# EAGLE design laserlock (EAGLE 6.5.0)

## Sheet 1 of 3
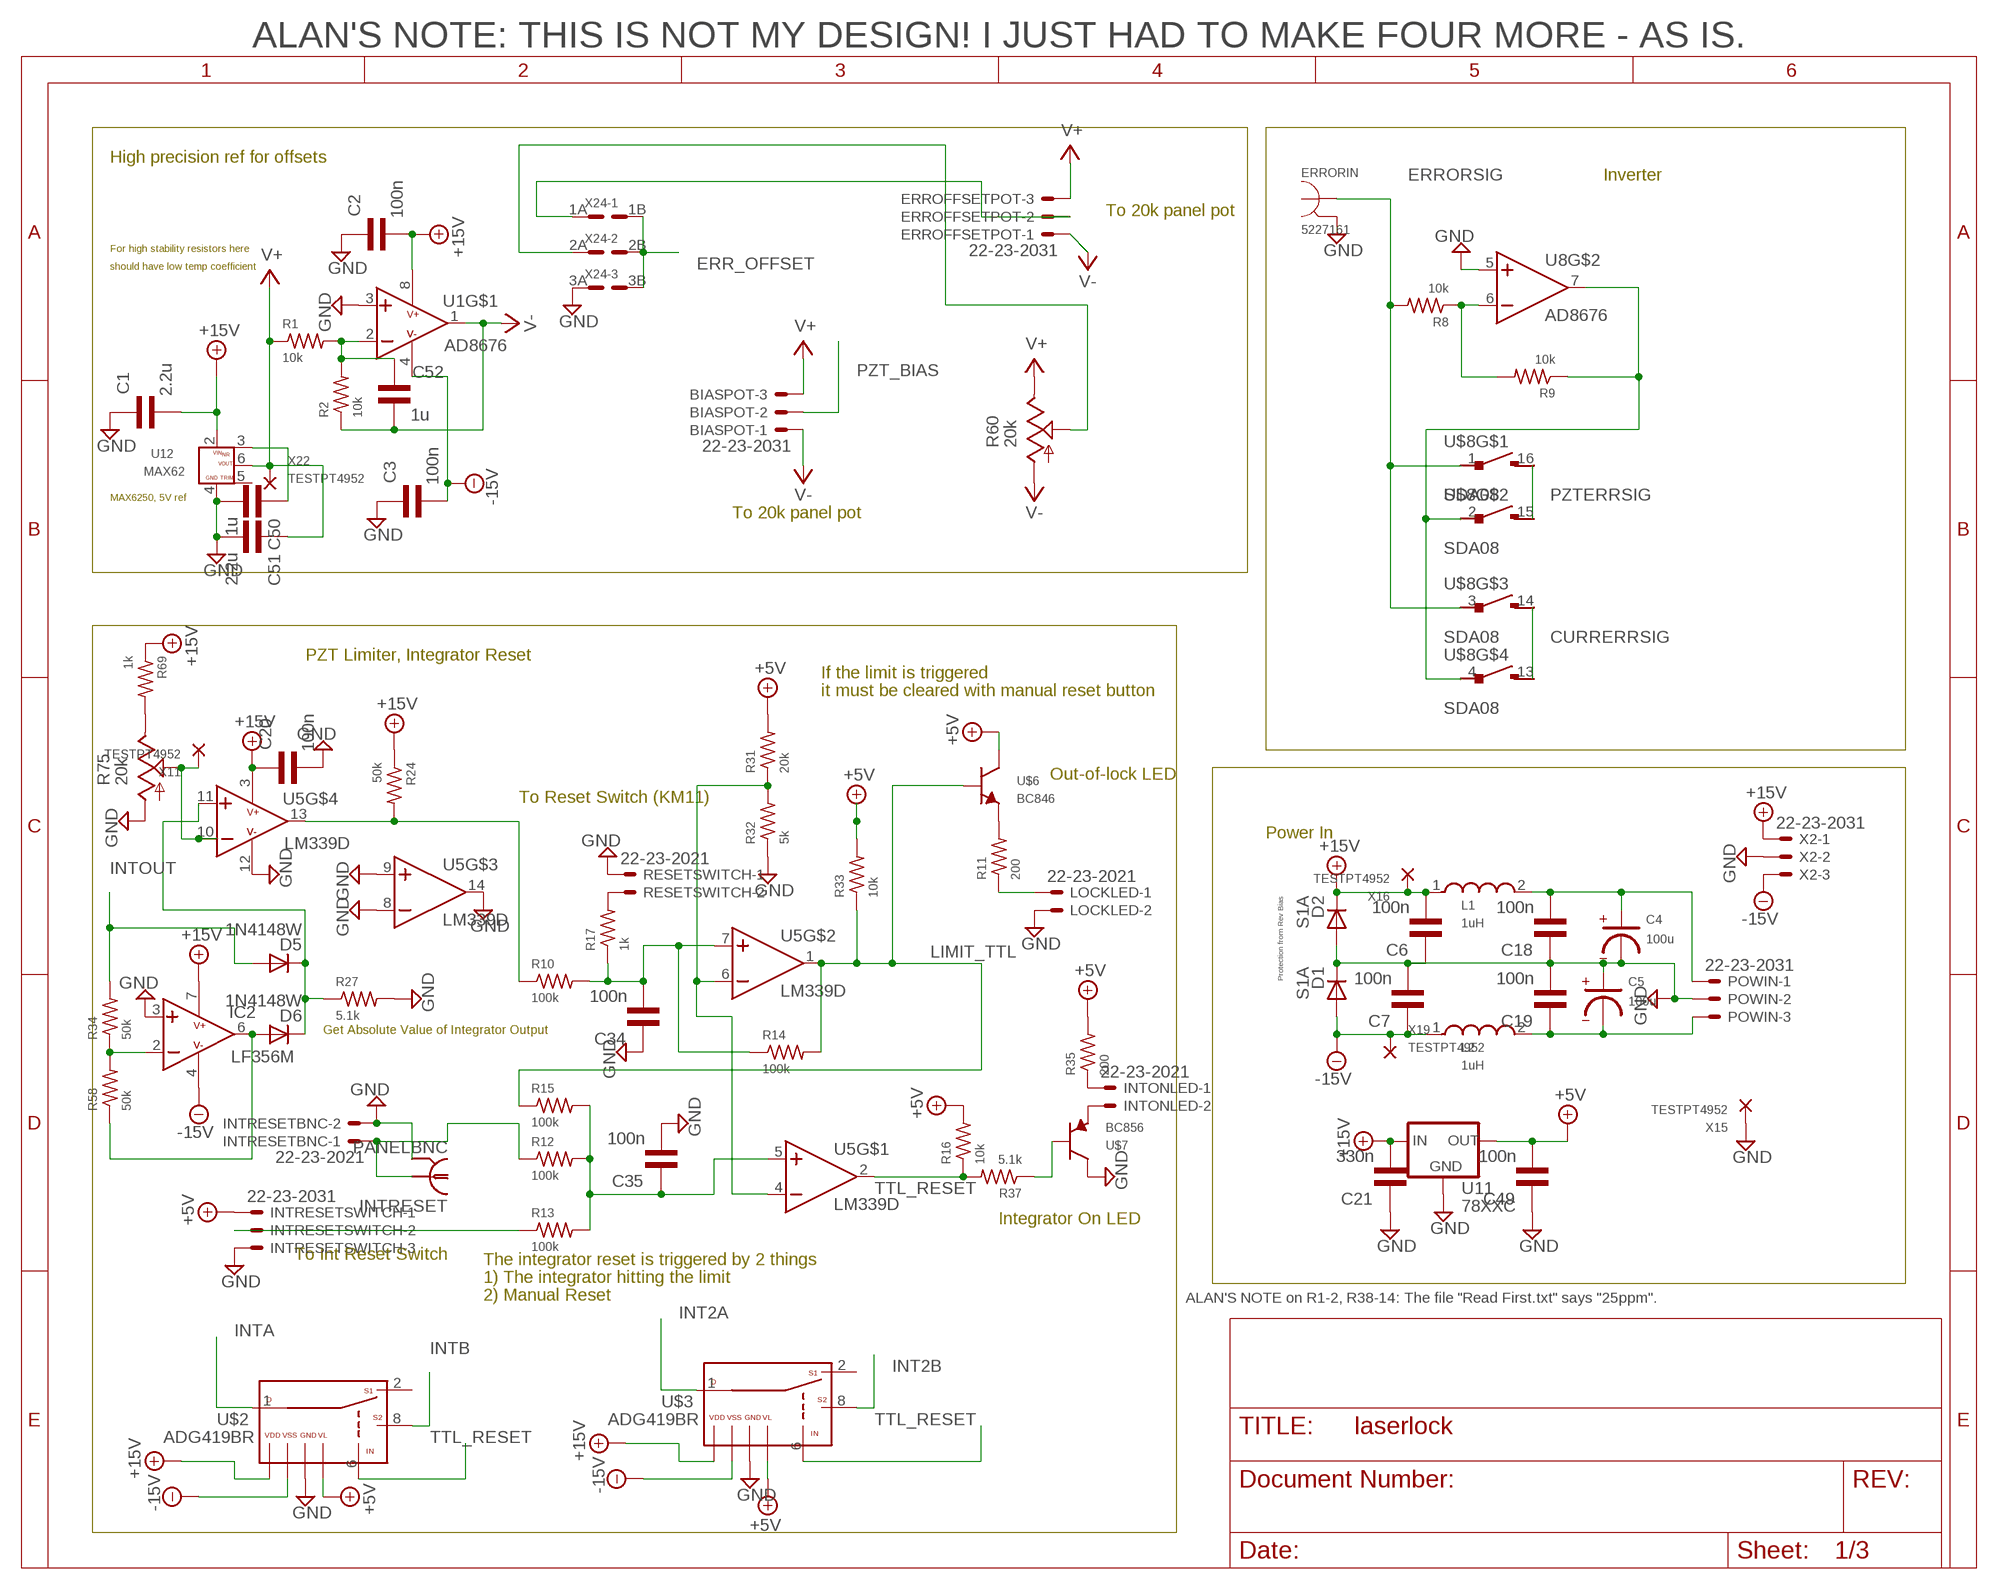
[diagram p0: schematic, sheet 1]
INTRESET (PANELBNC): DISTRIBUTOR: L-COM; PARTNUM: BAC1503

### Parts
BIASPOT  22-23-2031  [22-23-2031]
C1  2.2u  CAP0805  [0805]
C2  100n  CAP0805  [0805]
C3  100n  CAP0805  [0805]
C4  100u  CAPPOLRADIAL-0.1SPACING  [ELECCAPTH1]
C5  100u  CAPPOLRADIAL-0.1SPACING  [ELECCAPTH1]
C6  100n  CAP0805  [0805]
C7  100n  CAP0805  [0805]
C18  100n  CAP0805  [0805]
C19  100n  CAP0805  [0805]
C20  100n  CAP0805  [0805]
C21  330n  CAP0805  [0805]
C34  100n  CAP0805  [0805]
C35  100n  CAP0805  [0805]
C49  100n  CAP0805  [0805]
C50  1u  CAP0805  [0805]
C51  2.2u  CAP0805  [0805]
C52  1u  CAP0805  [0805]
D1  S1A  [DO-214AC]
D2  S1A  [DO-214AC]
D5  1N4148W  [SOD-323F]
D6  1N4148W  [SOD-323F]
ERROFFSETPOT  22-23-2031  [22-23-2031]
ERRORIN  5227161  [5227161]
IC2  LF356M  [SO08]
INTONLED  22-23-2021  [22-23-2021]
INTRESETBNC  22-23-2021  [22-23-2021]
INTRESETSWITCH  22-23-2031  [22-23-2031]
L1  1uH  INDUCTOR0805  [0805]
L2  1uH  INDUCTOR0805  [0805]
LOCKLED  22-23-2021  [22-23-2021]
POWIN  22-23-2031  [22-23-2031]
R1  10k  RESISTOR0805  [0805]
R2  10k  RESISTOR0805  [0805]
R8  10k  RESISTOR0805  [0805]
R9  10k  RESISTOR0805  [0805]
R10  100k  RESISTOR0805  [0805]
R11  200  RESISTOR1210  [1210]
R12  100k  RESISTOR0805  [0805]
R13  100k  RESISTOR0805  [0805]
R14  100k  RESISTOR0805  [0805]
R15  100k  RESISTOR0805  [0805]
R16  10k  RESISTOR0805  [0805]
R17  1k  RESISTOR0805  [0805]
R24  50k  RESISTOR0805  [0805]
R27  5.1k  RESISTOR0805  [0805]
R31  20k  RESISTOR0805  [0805]
R32  5k  RESISTOR0805  [0805]
R33  10k  RESISTOR0805  [0805]
R34  50k  RESISTOR0805  [0805]
R35  200  RESISTOR1210  [1210]
R37  5.1k  RESISTOR0805  [0805]
R58  50k  RESISTOR0805  [0805]
R60  20k  BITECH23B  [BITECH23B]
R69  1k  RESISTOR0805  [0805]
R75  20k  BITECH23B  [BITECH23B]
RESETSWITCH  22-23-2021  [22-23-2021]
U1  AD8676  [SO08]
U5  LM339D  [SO14]
U8  AD8676  [SO08]
U11  78XXC  [TO-220]
U12  MAX62  [SO08]
U$2  ADG419BR  [SO08]
U$3  ADG419BR  [SO08]
U$6  BC846  [SOT-23]
U$7  BC856  [SOT-23]
U$8  SDA08  [DIL16]
X2  22-23-2031  [22-23-2031]
X11  TESTPT4952  [TESTPT4952]
X15  TESTPT4952  [TESTPT4952]
X16  TESTPT4952  [TESTPT4952]
X19  TESTPT4952  [TESTPT4952]
X22  TESTPT4952  [TESTPT4952]
X24  HEADER2ROW3POS  [HEADER2ROW3POS]

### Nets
+5V: C49.2 INTRESETSWITCH.1 R16.2 R31.2 R33.2 R35.P$2 U11.3(OUT) U$2.5(VL) U$3.5(VL) U$6.3(C)
+15V: C1.2 C2.2 C6.2 C20.1 C21.2 D2.1(CATHODE) IC2.7(V+) L1.1 R24.1 R69.1 U1.8(V+) U5.3(V+) U11.1(IN) U12.2(VIN) U$2.4(V+) U$3.4(V+) X2.1 X16.P$1 ; also sheet 2,3
-15V: C3.2 C7.1 D1.2(ANODE) IC2.4(V-) L2.1 U1.4(V-) U$2.7(V-) U$3.7(V-) X2.3 X19.P$1 ; also sheet 2,3
CURRERRSIG: U$8.13 U$8.14 ; also sheet 3
ERR_OFFSET: X24.1B X24.2B X24.3B ; also sheet 2
ERRORSIG: ERRORIN.INCOND R8.2 U$8.1 U$8.3
GND: C1.1 C2.1 C3.1 C4.MINUS C5.PLUS C6.1 C7.2 C18.1 C19.2 C20.2 C21.1 C34.1 C35.2 C49.1 C50.2 C51.2 D1.1(CATHODE) D2.2(ANODE) ERRORIN.OUTCOND IC2.3(IN+) INTRESETBNC.2 INTRESETSWITCH.3 LOCKLED.2 POWIN.2 R27.2 R32.1 R75.1(A) RESETSWITCH.1 U1.3(IN+) U5.8(IN-) U5.9(IN+) U5.12(V-) U5.14(OUT) U8.5(IN+) U11.2(GND) U12.4(GND) U$2.3(GND) U$3.3(GND) U$7.3(C) X2.2 X15.P$1 X24.3A ; also sheet 2,3
INT2A: U$3.1(D) ; also sheet 2
INT2B: U$3.8(S2) ; also sheet 2
INTA: U$2.1(D) ; also sheet 2
INTB: U$2.8(S2) ; also sheet 2
INTOUT: D5.1(ANODE) R34.2 ; also sheet 2
LIMIT_TTL: R14.2 R15.1 R33.1 U5.1(OUT) U$6.1(B)
N$2: C52.1 R1.2 R2.2 U1.2(IN-)
N$5: R69.2 R75.3(E)
N$10: INTRESETBNC.1 R12.1
N$11: INTONLED.2 U$7.2(E)
N$12: INTRESETSWITCH.2 R13.1
N$13: R37.1 U$7.1(B)
N$14: C50.1 U12.3(NR)
N$15: R8.1 R9.2 U8.6(IN-)
N$16: C34.2 R10.2 R14.1 R17.1 U5.7(IN+)
N$17: C35.1 R12.2 R13.2 R15.2 U5.5(IN+)
N$18: R17.2 RESETSWITCH.2
N$37: ERROFFSETPOT.2 X24.1A
N$39: R9.1 U8.7(OUT) U$8.2 U$8.4
N$40: R10.1 R24.2 U5.13(OUT)
N$41: R31.1 R32.2 U5.4(IN-) U5.6(IN-)
N$42: R11.P$2 U$6.2(E)
N$43: R75.2(S) U5.10(IN-) X11.P$1
N$45: LOCKLED.1 R11.P$1
N$49: C5.MINUS C19.1 L2.2 POWIN.3
N$50: C4.PLUS C18.2 L1.2 POWIN.1
N$51: D5.2(CATHODE) D6.2(CATHODE) R27.1 U5.11(IN+)
N$54: R60.2(S) X24.2A
N$70: INTONLED.1 R35.P$1
N$80: IC2.2(IN-) R34.1 R58.2
N$81: D6.1(ANODE) IC2.6(OUT) R58.1
PZT_BIAS: BIASPOT.2 ; also sheet 2
PZTERRSIG: U$8.15 U$8.16 ; also sheet 2
TTL_RESET: R16.1 R37.2 U5.2(OUT) U$2.6(IN) U$3.6(IN)
V+: BIASPOT.3 C51.1 ERROFFSETPOT.3 R1.1 R60.3(E) U12.6(VO) X22.P$1
V-: BIASPOT.1 C52.2 ERROFFSETPOT.1 R2.1 R60.1(A) U1.1(OUT)
Unconnected: U12.5(TRIM) U$2.2(S1) U$3.2(S1)

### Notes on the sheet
- ALAN'S NOTE: THIS IS NOT MY DESIGN! I JUST HAD TO MAKE FOUR MORE - AS IS.
- High precision ref for offsets
- Inverter
- To 20k panel pot
- For high stability resistors here
- should have low temp coefficient
- MAX6250, 5V ref
- To 20k panel pot
- PZT Limiter, Integrator Reset
- If the limit is triggered
- it must be cleared with manual reset button
- Out-of-lock LED
- To Reset Switch (KM11)
- Power In
- Protection from Rev Bias
- Get Absolute Value of Integrator Output
- Integrator On LED
- To Int Reset Switch
- The integrator reset is triggered by 2 things
- 1) The integrator hitting the limit
- ALAN'S NOTE on R1-2, R38-14: The file "Read First.txt" says "25ppm".
- 2) Manual Reset

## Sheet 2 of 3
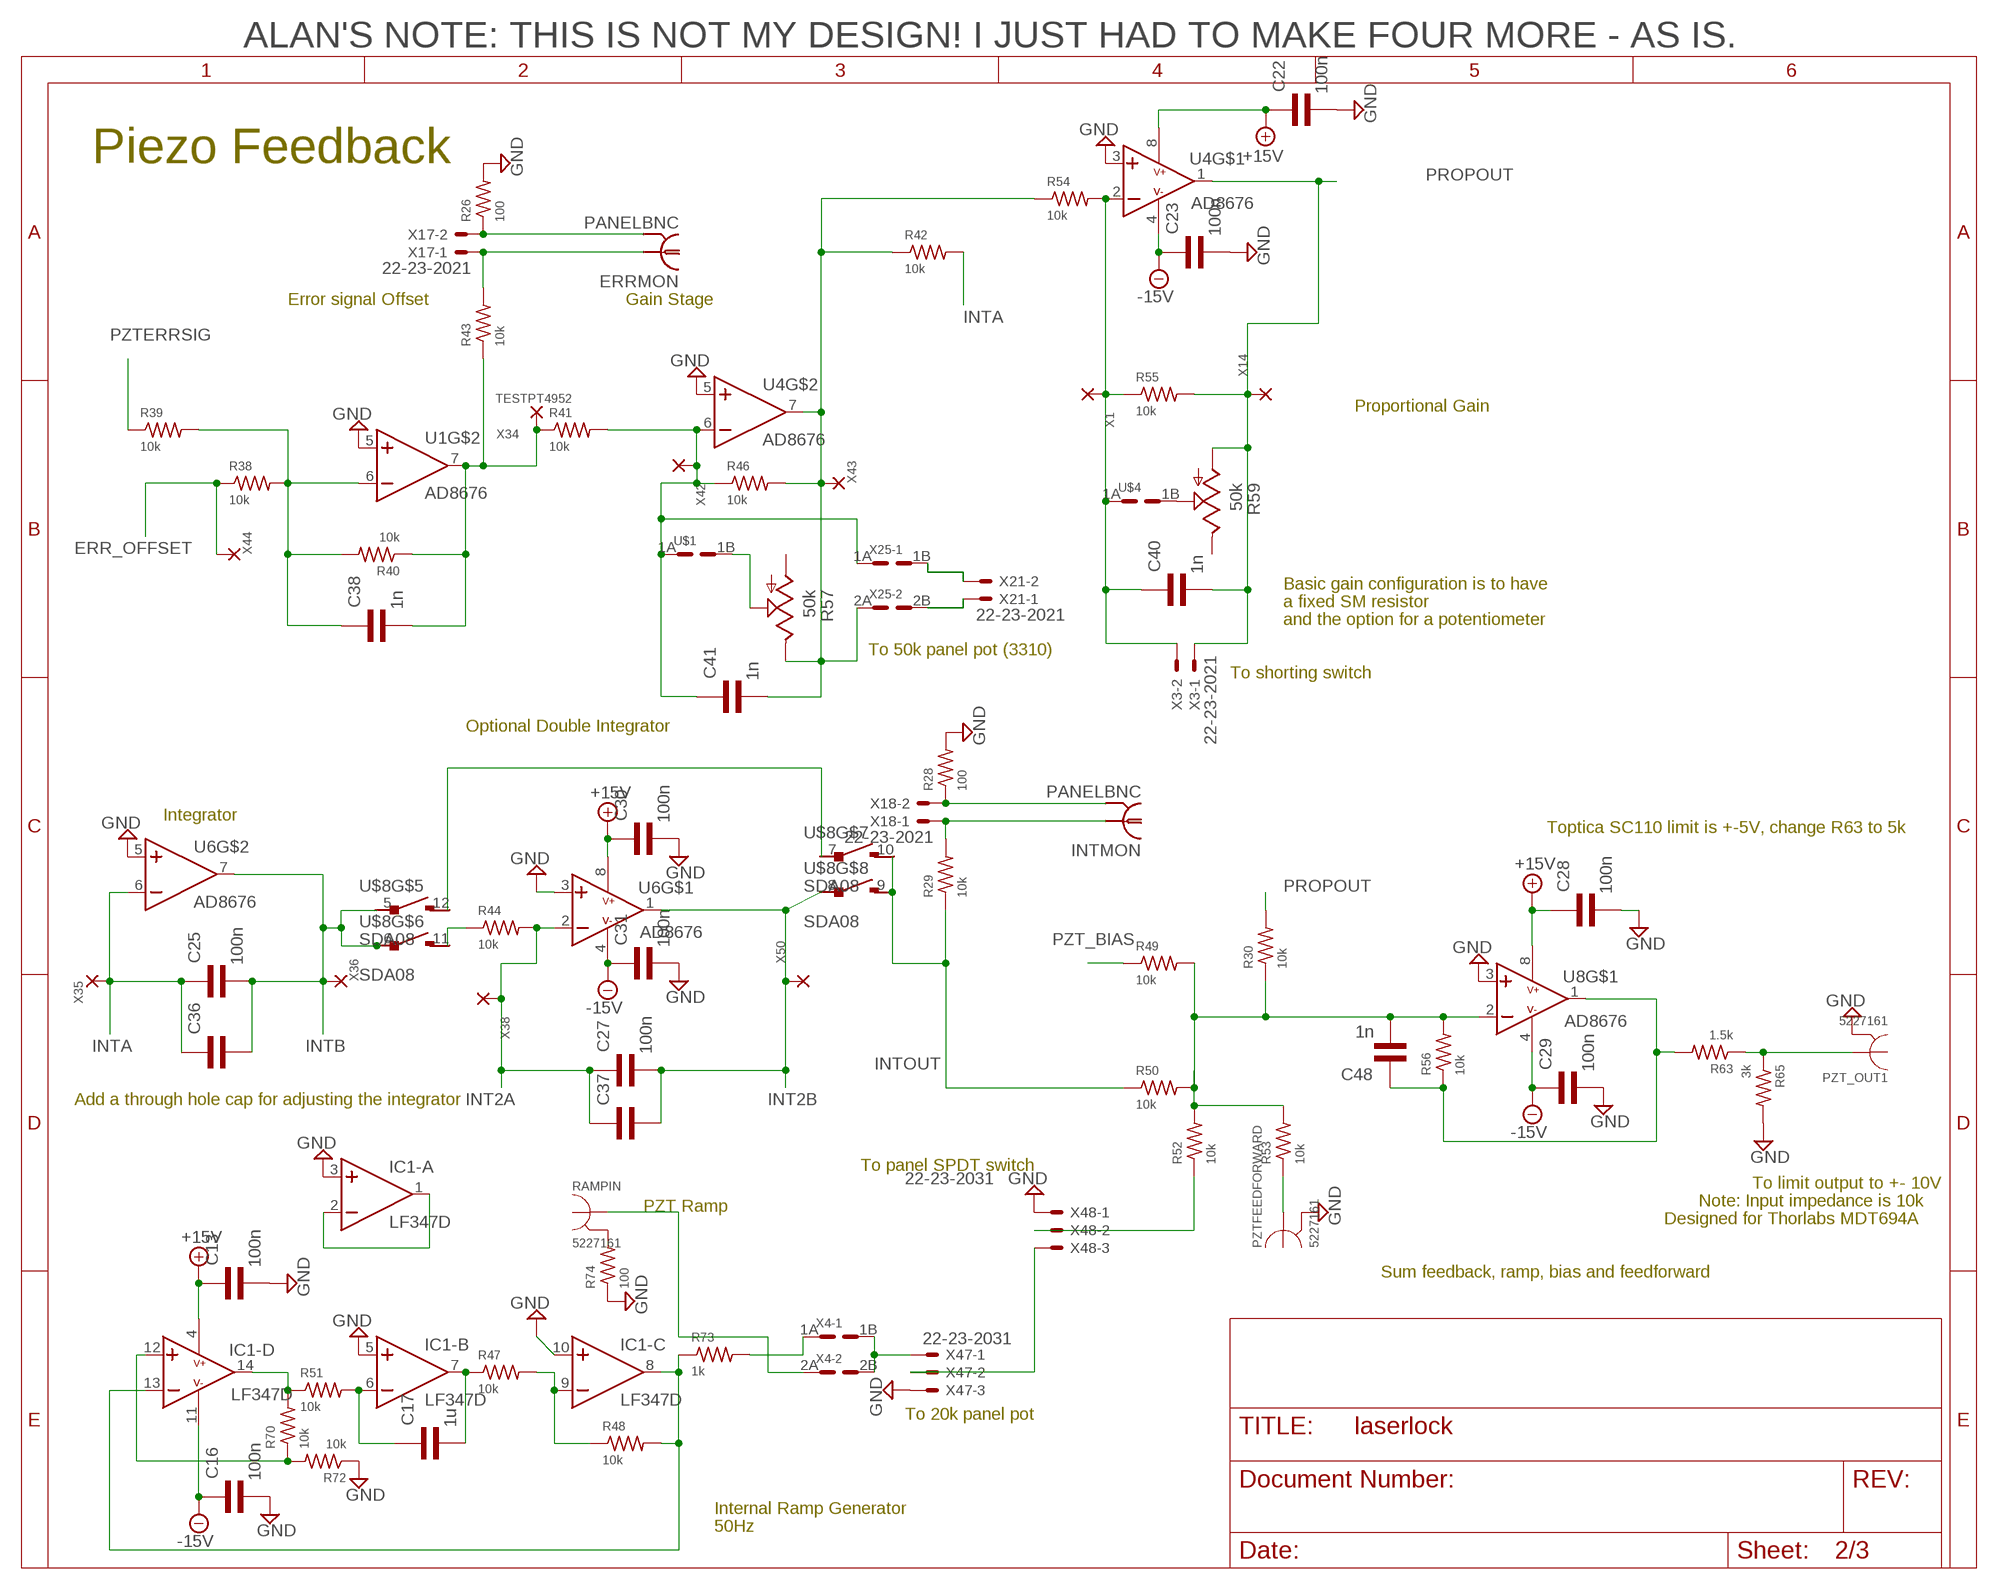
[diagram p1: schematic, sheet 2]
ERRMON (PANELBNC): DISTRIBUTOR: L-COM; PARTNUM: BAC1503
INTMON (PANELBNC): DISTRIBUTOR: L-COM; PARTNUM: BAC1503

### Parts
C13  100n  CAP0805  [0805]
C16  100n  CAP0805  [0805]
C17  1u  CAP0805  [0805]
C22  100n  CAP0805  [0805]
C23  100n  CAP0805  [0805]
C25  100n  CAP0805  [0805]
C27  100n  CAP0805  [0805]
C28  100n  CAP0805  [0805]
C29  100n  CAP0805  [0805]
C30  100n  CAP0805  [0805]
C31  100n  CAP0805  [0805]
C36  CAPTH1  [TH1]
C37  CAPTH1  [TH1]
C38  1n  CAP0805  [0805]
C40  1n  CAP0805  [0805]
C41  1n  CAP0805  [0805]
C48  1n  CAP0805  [0805]
IC1  LF347D  [SO14]
PZT_OUT1  5227161  [5227161]
PZTFEEDFORWARD  5227161  [5227161]
R26  100  RESISTOR0805  [0805]
R28  100  RESISTOR0805  [0805]
R29  10k  RESISTOR0805  [0805]
R30  10k  RESISTOR0805  [0805]
R38  10k  RESISTOR0805  [0805]
R39  10k  RESISTOR0805  [0805]
R40  10k  RESISTOR0805  [0805]
R41  10k  RESISTOR0805  [0805]
R42  10k  RESISTOR0805  [0805]
R43  10k  RESISTOR0805  [0805]
R44  10k  RESISTOR0805  [0805]
R46  10k  RESISTOR0805  [0805]
R47  10k  RESISTOR0805  [0805]
R48  10k  RESISTOR0805  [0805]
R49  10k  RESISTOR0805  [0805]
R50  10k  RESISTOR0805  [0805]
R51  10k  RESISTOR0805  [0805]
R52  10k  RESISTOR0805  [0805]
R53  10k  RESISTOR0805  [0805]
R54  10k  RESISTOR0805  [0805]
R55  10k  RESISTOR0805  [0805]
R56  10k  RESISTOR0805  [0805]
R57  50k  BITECH23B  [BITECH23B]
R59  50k  BITECH23B  [BITECH23B]
R63  1.5k  RESISTOR0805  [0805]
R65  3k  RESISTOR0805  [0805]
R70  10k  RESISTOR0805  [0805]
R72  10k  RESISTOR0805  [0805]
R73  1k  RESISTOR0805  [0805]
R74  100  RESISTOR0805  [0805]
RAMPIN  5227161  [5227161]
U4  AD8676  [SO08]
U6  AD8676  [SO08]
U$1  HEADER2ROW1POS  [HEADER2ROW1POS]
U$4  HEADER2ROW1POS  [HEADER2ROW1POS]
X1  TESTPT4952  [TESTPT4952]
X3  22-23-2021  [22-23-2021]
X4  HEADER2ROW2POS  [HEADER2ROW2POS]
X14  TESTPT4952  [TESTPT4952]
X17  22-23-2021  [22-23-2021]
X18  22-23-2021  [22-23-2021]
X21  22-23-2021  [22-23-2021]
X25  HEADER2ROW2POS  [HEADER2ROW2POS]
X34  TESTPT4952  [TESTPT4952]
X35  TESTPT4952  [TESTPT4952]
X36  TESTPT4952  [TESTPT4952]
X38  TESTPT4952  [TESTPT4952]
X42  TESTPT4952  [TESTPT4952]
X43  TESTPT4952  [TESTPT4952]
X44  TESTPT4952  [TESTPT4952]
X47  22-23-2031  [22-23-2031]
X48  22-23-2031  [22-23-2031]
X50  TESTPT4952  [TESTPT4952]

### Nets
+15V: C13.1 C22.1 C28.1 C30.1 IC1.4(-D:V+) U4.8(V+) U6.8(V+) U8.8(V+) ; also sheet 1,3
-15V: C16.1 C23.1 C29.1 C31.1 IC1.11(-D:V-) U4.4(V-) U6.4(V-) U8.4(V-) ; also sheet 1,3
ERR_OFFSET: R38.1 X44.P$1 ; also sheet 1
GND: C13.2 C16.2 C22.2 C23.2 C28.2 C29.2 C30.2 C31.2 IC1.3(-A:IN+) IC1.5(-B:IN+) IC1.10(-C:IN+) PZT_OUT1.OUTCOND PZTFEEDFORWARD.OUTCOND R26.2 R28.2 R65.2 R72.1 R74.1 U1.5(IN+) U4.3(IN+) U4.5(IN+) U6.3(IN+) U6.5(IN+) U8.3(IN+) X47.3 X48.1 ; also sheet 1,3
INT2A: C27.1 C37.P$1 R44.2 U6.2(IN-) X38.P$1 ; also sheet 1
INT2B: C27.2 C37.P$2 U6.1(OUT) U$8.8 X50.P$1 ; also sheet 1
INTA: C25.1 C36.P$1 R42.2 U6.6(IN-) X35.P$1 ; also sheet 1
INTB: C25.2 C36.P$2 U6.7(OUT) U$8.5 U$8.6 X36.P$1 ; also sheet 1
INTOUT: R29.1 R50.1 U$8.9 U$8.10 ; also sheet 1
N$21: C41.2 R42.1 R46.2 R54.1 R57.3(E) U4.7(OUT) X25.2A X43.P$1
N$28: R26.1 X17.2
N$29: R29.2 X18.1
N$30: X21.2 X25.1B
N$33: IC1.1(-A:OUT) IC1.2(-A:IN-)
N$34: C17.2 IC1.7(-B:OUT) R47.1
N$35: R43.2 X17.1
N$36: R28.1 X18.2
N$38: X21.1 X25.2B
N$46: C40.1 R54.2 R55.1 U4.2(IN-) U$4.1A X1.P$1 X3.2
N$47: C38.1 R38.2 R39.2 R40.2 U1.6(IN-)
N$48: C38.2 R40.1 R41.1 R43.1 U1.7(OUT) X34.P$1
N$53: U$8.7 U$8.12
N$55: R44.1 U$8.11
N$56: X47.2 X48.3
N$59: C41.1 R41.2 R46.1 U4.6(IN-) U$1.1A X25.1A X42.P$1
N$60: R57.2(S) U$1.1B
N$62: IC1.9(-C:IN-) R47.2 R48.1
N$63: IC1.8(-C:OUT) IC1.13(-D:IN-) R48.2 R73.1
N$64: C17.1 IC1.6(-B:IN-) R51.2
N$65: X4.1B X4.2B X47.1
N$66: R59.2(S) U$4.1B
N$67: PZTFEEDFORWARD.INCOND R53.1
N$68: C48.2 R30.1 R49.2 R50.2 R52.2 R53.2 R56.2 U8.2(IN-)
N$69: R52.1 X48.2
N$72: C48.1 R56.1 R63.2 U8.1(OUT)
N$73: PZT_OUT1.INCOND R63.1 R65.1
N$75: IC1.14(-D:OUT) R51.1 R70.2
N$78: IC1.12(-D:IN+) R70.1 R72.2
N$82: RAMPIN.INCOND X4.2A
N$83: R73.2 X4.1A
N$84: R74.2 RAMPIN.OUTCOND
PROPOUT: C40.2 R30.2 R55.2 R59.1(A) U4.1(OUT) X3.1 X14.P$1
PZT_BIAS: R49.1 ; also sheet 1
PZTERRSIG: R39.1 ; also sheet 1
Unconnected: R57.1(A) R59.3(E)

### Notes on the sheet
- ALAN'S NOTE: THIS IS NOT MY DESIGN! I JUST HAD TO MAKE FOUR MORE - AS IS.
- Piezo Feedback
- Error signal Offset | Gain Stage
- Proportional Gain
- Basic gain configuration is to have
- a fixed SM resistor
- and the option for a potentiometer
- To 50k panel pot (3310)
- To shorting switch
- Optional Double Integrator
- Integrator | Toptica SC110 limit is +-5V, change R63 to 5k
- Add a through hole cap for adjusting the integrator
- To panel SPDT switch
- To limit output to +- 10V
- Note: Input impedance is 10k
- PZT Ramp | Designed for Thorlabs MDT694A
- Sum feedback, ramp, bias and feedforward
- To 20k panel pot
- Internal Ramp Generator
- 50Hz

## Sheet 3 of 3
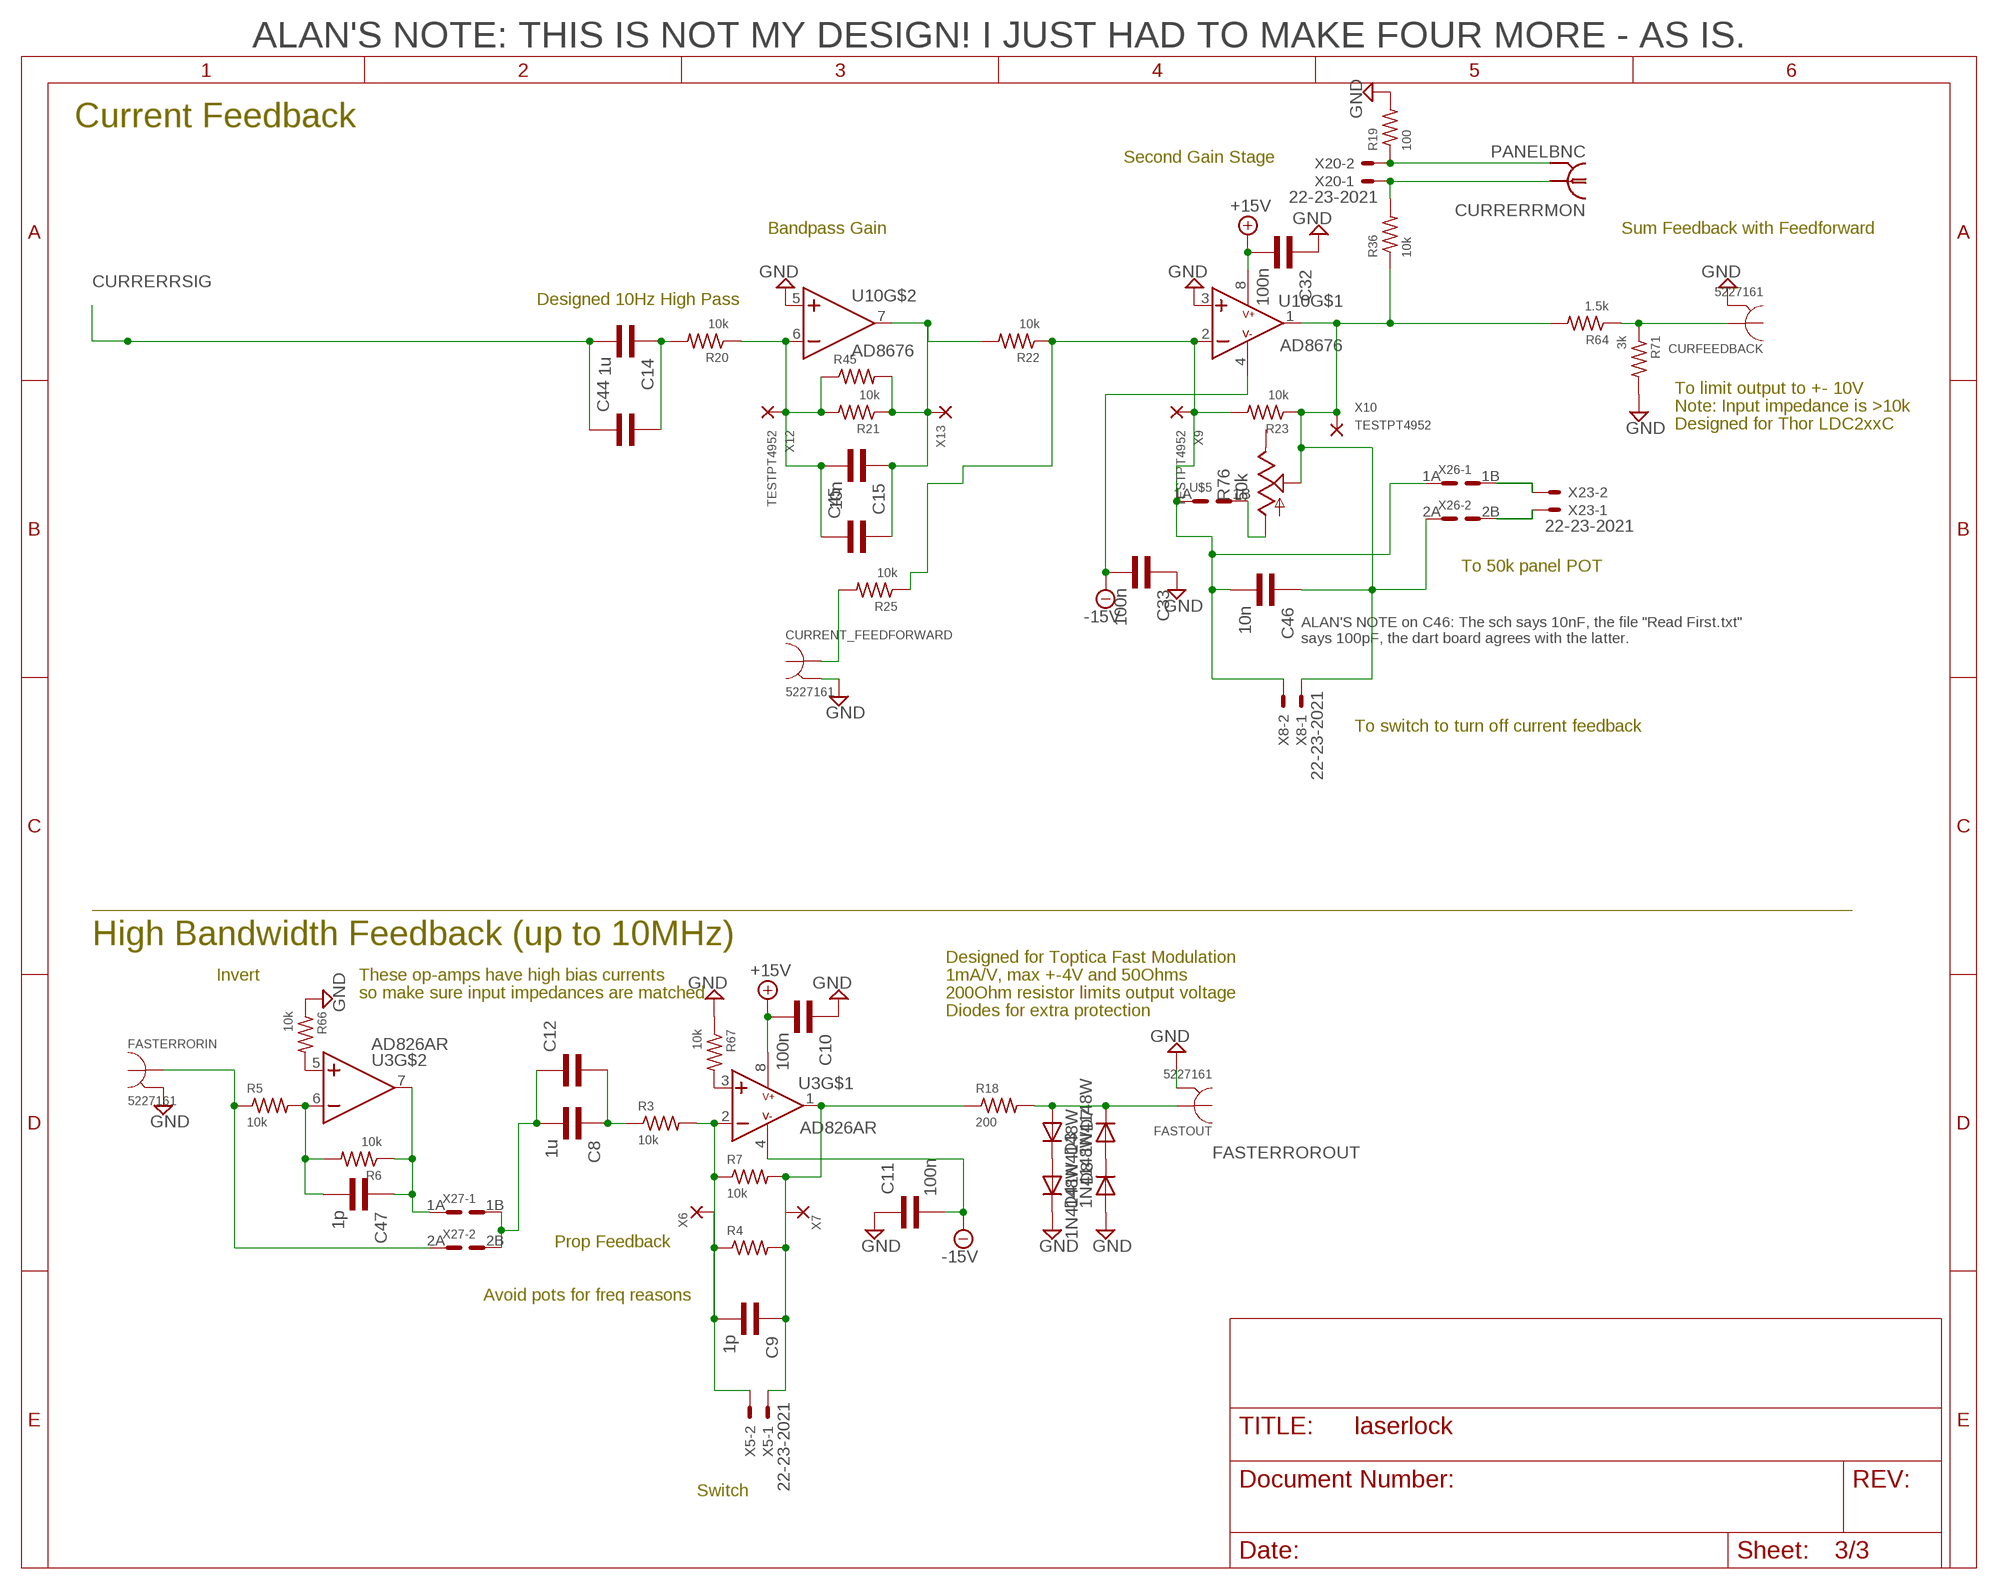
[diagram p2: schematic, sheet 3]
CURRERRMON (PANELBNC): DISTRIBUTOR: L-COM; PARTNUM: BAC1503

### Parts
C8  1u  CAP0805  [0805]
C9  1p  CAP0805  [0805]
C10  100n  CAP0805  [0805]
C11  100n  CAP0805  [0805]
C12  CAPTH1  [TH1]
C14  1u  CAP0805  [0805]
C15  10n  CAP0805  [0805]
C32  100n  CAP0805  [0805]
C33  100n  CAP0805  [0805]
C44  CAPTH1  [TH1]
C45  CAPTH1  [TH1]
C46  10n  CAP0805  [0805]
C47  1p  CAP0805  [0805]
CURFEEDBACK  5227161  [5227161]
CURRENT_FEEDFORWARD  5227161  [5227161]
D3  1N4148W  [SOD-323F]
D4  1N4148W  [SOD-323F]
D7  1N4148W  [SOD-323F]
D8  1N4148W  [SOD-323F]
FASTERRORIN  5227161  [5227161]
FASTOUT  5227161  [5227161]
R3  10k  RESISTOR0805  [0805]
R4  RESISTORTH1  [TH1]
R5  10k  RESISTOR0805  [0805]
R6  10k  RESISTOR0805  [0805]
R7  10k  RESISTOR0805  [0805]
R18  200  RESISTOR1210  [1210]
R19  100  RESISTOR0805  [0805]
R20  10k  RESISTOR0805  [0805]
R21  10k  RESISTOR0805  [0805]
R22  10k  RESISTOR0805  [0805]
R23  10k  RESISTOR0805  [0805]
R25  10k  RESISTOR0805  [0805]
R36  10k  RESISTOR0805  [0805]
R45  RESISTORTH1  [TH1]
R64  1.5k  RESISTOR0805  [0805]
R66  10k  RESISTOR0805  [0805]
R67  10k  RESISTOR0805  [0805]
R71  3k  RESISTOR0805  [0805]
R76  50k  BITECH23B  [BITECH23B]
U3  AD826AR  [SO08]
U10  AD8676  [SO08]
U$5  HEADER2ROW1POS  [HEADER2ROW1POS]
X5  22-23-2021  [22-23-2021]
X6  TESTPT4952  [TESTPT4952]
X7  TESTPT4952  [TESTPT4952]
X8  22-23-2021  [22-23-2021]
X9  TESTPT4952  [TESTPT4952]
X10  TESTPT4952  [TESTPT4952]
X12  TESTPT4952  [TESTPT4952]
X13  TESTPT4952  [TESTPT4952]
X20  22-23-2021  [22-23-2021]
X23  22-23-2021  [22-23-2021]
X26  HEADER2ROW2POS  [HEADER2ROW2POS]
X27  HEADER2ROW2POS  [HEADER2ROW2POS]

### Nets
+15V: C10.2 C32.2 U3.8(V+) U10.8(V+) ; also sheet 1,2
-15V: C11.2 C33.2 U3.4(V-) U10.4(V-) ; also sheet 1,2
CURRERRSIG: C14.2 C44.P$1 ; also sheet 1
FASTERROR-: C8.2 C12.P$1 X27.1B X27.2B
FASTERROROUT: D3.1(ANODE) D7.2(CATHODE) FASTOUT.INCOND R18.P$2
GND: C10.1 C11.1 C32.1 C33.1 CURFEEDBACK.OUTCOND CURRENT_FEEDFORWARD.OUTCOND D4.2(CATHODE) D8.1(ANODE) FASTERRORIN.OUTCOND FASTOUT.OUTCOND R19.2 R66.1 R67.1 R71.2 U10.3(IN+) U10.5(IN+) ; also sheet 1,2
N$1: C9.2 R3.2 R4.P$1 R7.1 U3.2(IN-) X5.2 X6.P$1
N$3: C8.1 C12.P$2 R3.1
N$4: C46.2 R22.1 R23.2 R25.1 U10.2(IN-) U$5.1A X8.2 X9.P$1 X26.1A
N$6: C9.1 R4.P$2 R7.2 R18.P$1 U3.1(OUT) X5.1 X7.P$1
N$7: C47.2 R5.2 R6.2 U3.6(IN-)
N$8: FASTERRORIN.INCOND R5.1 X27.2A
N$9: C47.1 R6.1 U3.7(OUT) X27.1A
N$19: C15.1 C45.P$2 R21.1 R22.2 R45.P$2 U10.7(OUT) X13.P$1
N$20: C46.1 R23.1 R36.1 R64.2 R76.2(S) U10.1(OUT) X8.1 X10.P$1 X26.2A
N$22: C14.1 C44.P$2 R20.2
N$23: C15.2 C45.P$1 R20.1 R21.2 R45.P$1 U10.6(IN-) X12.P$1
N$24: D3.2(CATHODE) D4.1(ANODE)
N$25: D7.1(ANODE) D8.2(CATHODE)
N$26: R19.1 X20.2
N$27: CURRENT_FEEDFORWARD.INCOND R25.2
N$31: R76.1(A) U$5.1B
N$32: R36.2 X20.1
N$44: X23.2 X26.1B
N$52: X23.1 X26.2B
N$74: CURFEEDBACK.INCOND R64.1 R71.1
N$76: R66.2 U3.5(IN+)
N$77: R67.2 U3.3(IN+)
Unconnected: R76.3(E)

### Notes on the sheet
- ALAN'S NOTE: THIS IS NOT MY DESIGN! I JUST HAD TO MAKE FOUR MORE - AS IS.
- Current Feedback
- Second Gain Stage
- Bandpass Gain | Sum Feedback with Feedforward
- Designed 10Hz High Pass
- To limit output to +- 10V
- Note: Input impedance is >10k
- Designed for Thor LDC2xxC
- To 50k panel POT
- ALAN'S NOTE on C46: The sch says 10nF, the file "Read First.txt"
  says 100pF, the dart board agrees with the latter.
- To switch to turn off current feedback
- High Bandwidth Feedback (up to 10MHz)
- Designed for Toptica Fast Modulation
- Invert | These op-amps have high bias currents | 1mA/V, max +-4V and 50Ohms
- so make sure input impedances are matched | 200Ohm resistor limits output voltage
- Diodes for extra protection
- Prop Feedback
- Avoid pots for freq reasons
- Switch

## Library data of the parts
BIASPOT ERROFFSETPOT INTRESETSWITCH POWIN X2 X47 X48 = dcmckaylib:22-23-2031: .100" (2.54mm) Center Header - 3 Pin
C1-C3 C6-C23 C25 C27-C38 C40 C41 C44-C52 = dcmckaylib:CAP?: Standard Cap
C4 C5 = dcmckaylib:CAPPOL?: Polarized Capacitor. Can be either aluminum or tantalum electrolytic. Use appropriate package depending on the type (and capacitance)
CURFEEDBACK CURRENT_FEEDFORWARD ERRORIN FASTERRORIN FASTOUT PZT_OUT1 PZTFEEDFORWARD RAMPIN = dcmckaylib:5227161: Right Angle 50Ohm PCB BNC Connector. DigiKey Part #A32258-ND.
D1 D2 = dcmckaylib:S1A: 1A Rectifier Diode
D3-D8 = dcmckaylib:1N4148?: Small signal diode
IC1 = dcmckaylib:LF347?: Quad FET Op-Amp with 4MHz Bandwidth Low input bias current Moderate voltage noise and input voltage offset
IC2 = dcmckaylib:LF356?: LF356 Op Amp, National Semiconductor
INTONLED INTRESETBNC LOCKLED RESETSWITCH X3 X5 X8 X17 X18 X20 X21 X23 = dcmckaylib:22-23-2021: .100" (2.54mm) Center Header - 2 Pin
L1 L2 = dcmckaylib:INDUCTOR?: Inductor
R1-R56 R58 R63-R67 R69-R74 = dcmckaylib:RESISTOR?: Standard resistor. Packages starting in "TH" are through hole.
R57 R59 R60 R75 R76 = dcmckaylib:BITECH23?: Trim POT from BITECH Newark Part # 63M1857 (20k), 63M1861 (50k)
U1 U4 U6 U8 U10 = dcmckaylib:AD8676
U3 = dcmckaylib:AD826?: High speed (50MHz) dual op-amp 15nV/Hz^(0.5) voltage noise, 1.5pA/Hz^(0.5) current noise 15nA offset current (10uA bias)
U5 = dcmckaylib:LM339?: Quad Comparator. Same as LM239/2901.
U11 = dcmckaylib:78XX?: Voltage Regulator
U12 = dcmckaylib:MAX62*?: Precision Voltage Reference
U$1 U$4 U$5 = dcmckaylib:HEADER2ROW1POS
U$2 U$3 = dcmckaylib:ADG419?
U$6 = dcmckaylib:BC846: Surface Mount NPN 100mA max 45V C-E
U$7 = dcmckaylib:BC856: PNP 100mA ~100 gain
U$8 = dcmckaylib:SDA08
X1 X6 X7 X9-X16 X19 X22 X34-X36 X38 X42-X44 X50 = dcmckaylib:TESTPT?
X4 X25-X27 = dcmckaylib:HEADER2ROW2POS: Standard 0.1" 2x2 header
X24 = dcmckaylib:HEADER2ROW3POS

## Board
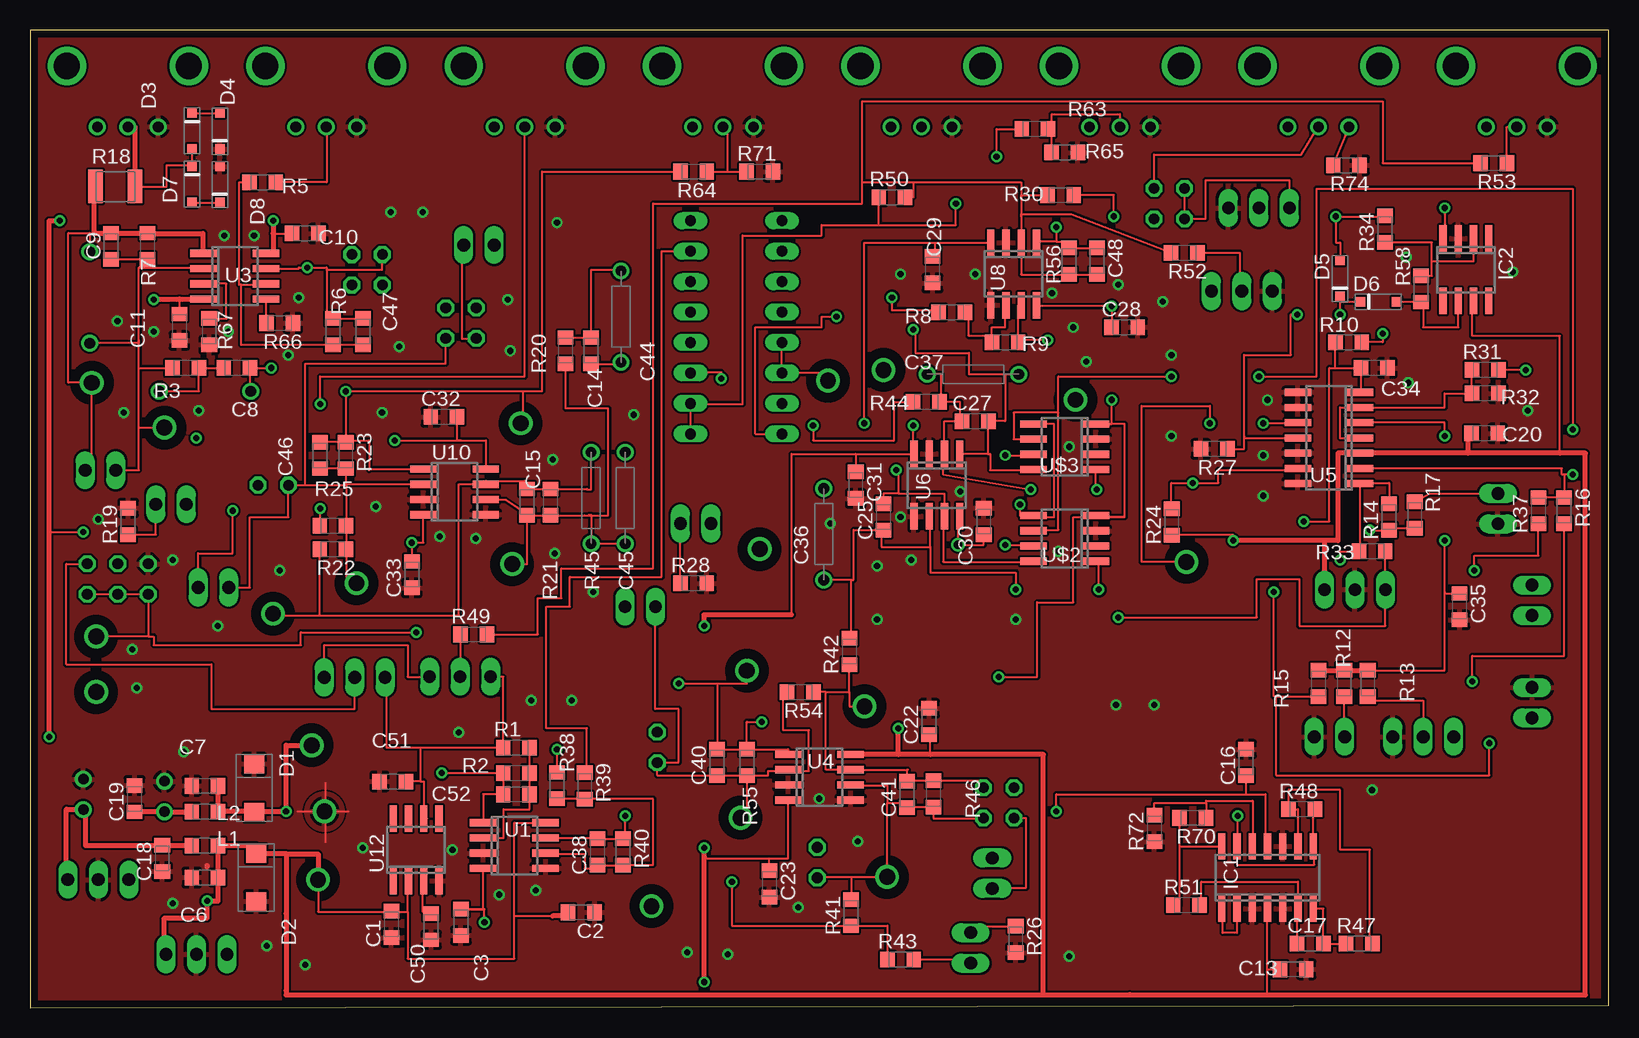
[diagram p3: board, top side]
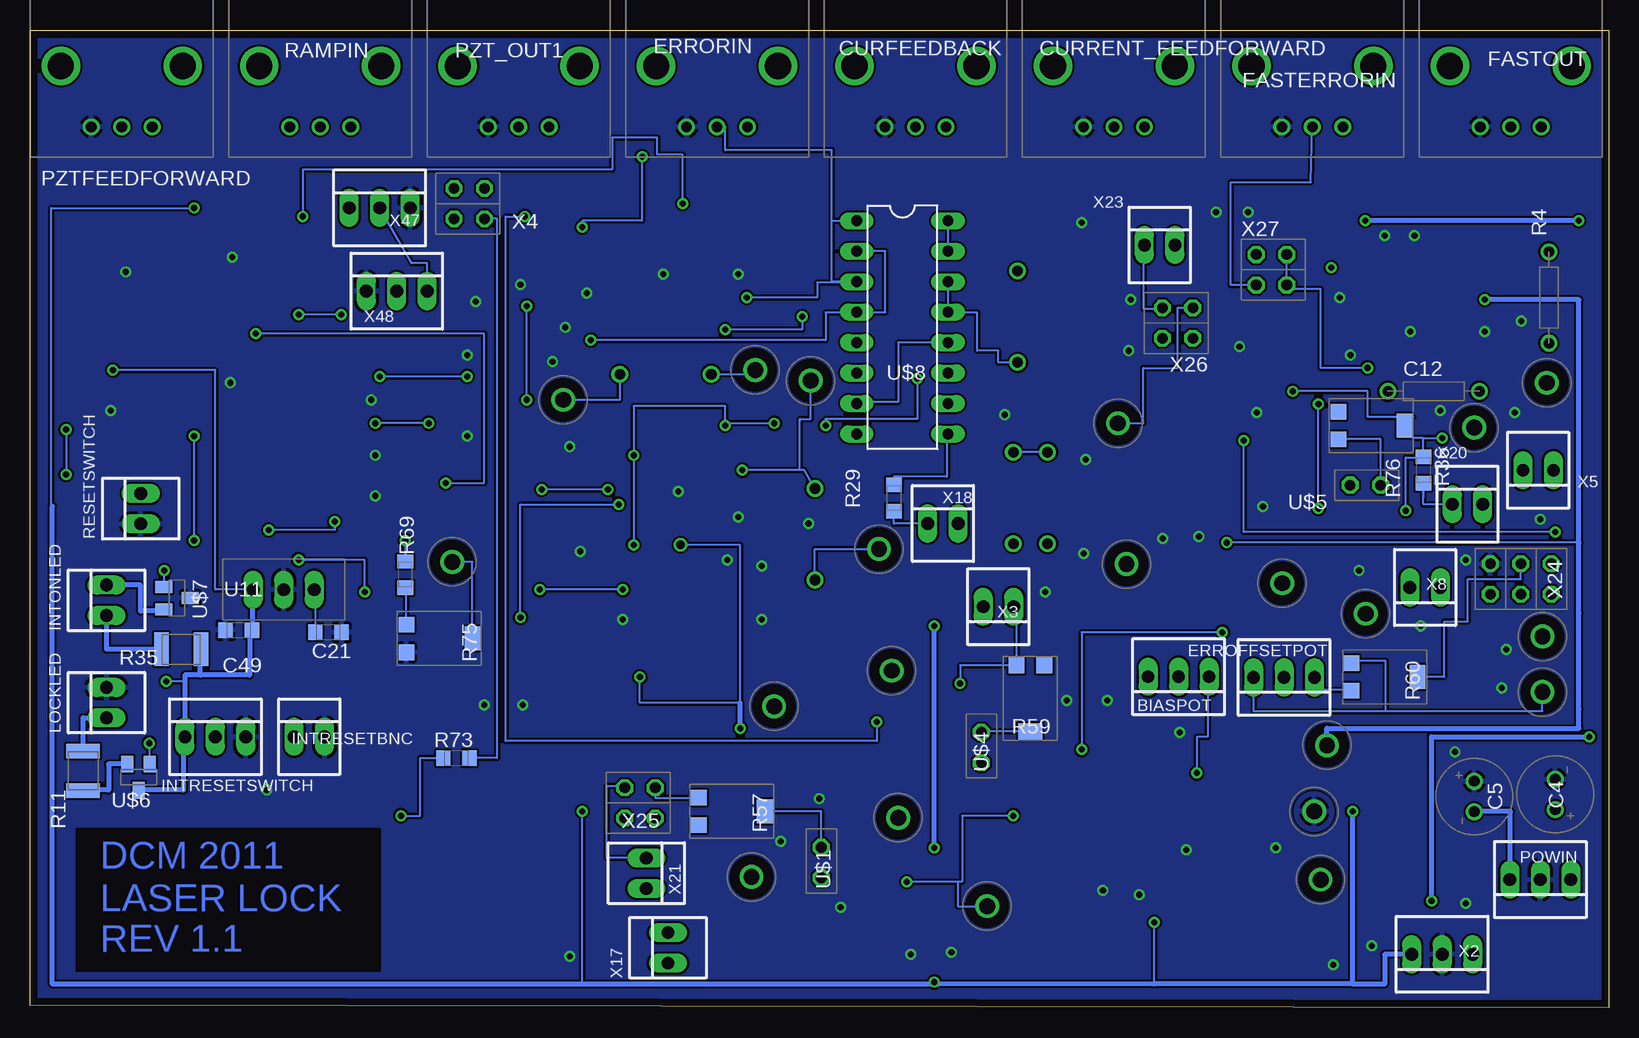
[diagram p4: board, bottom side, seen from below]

Size 131.55 x 81.51 mm. Coordinates in mm from the lower left corner, seen from the top.
Outline: 0,0 131.55,0.18 131.55,81.51 0,81.51 0,0
Copper layers (1+16): Top 0.035mm / dielectric 1.5mm / Bottom 0.035mm
Design rules "DRC standard check": minimum track width 7mil, minimum drill 20mil, track to track 7mil, track to pad 7mil, pad to pad 7mil, via to via 7mil, smd to smd 0mil, copper to edge 25mil, drill to drill 8mil, minimum pad ring 10mil, minimum via ring 8mil, stop-mask expansion 4mil, vias tented up to drill 0mil, thermal gap 10mil
bRestrict: 4 lines

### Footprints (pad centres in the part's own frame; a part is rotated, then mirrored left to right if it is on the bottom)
22-23-2031 = drill 1.067 long: 1 -2.54,0; 2 0,0; 3 2.54,0
0805 = smd 1.2 x 1.3: 1 -1.1,0; 2 1.1,0
ELECCAPTH1 = drill 0.889: MINUS 1.27,0; PLUS -1.27,0
TH1 = drill 0.889: P$1 -3.81,0; P$2 3.81,0
5227161 = drill 0.889: INCOND 1.27,0; OUTCOND -1.27,0; OUTCOND2 3.81,0 | drill 2.184: P$3 6.35,5.08; P$4 -3.81,5.08
DO-214AC = smd 1.55 x 1.67: 1 2,0; 2 -2,0
SOD-323F = smd 0.8 x 0.8: 1 -1.5,0; 2 1.5,0
SO14 = smd 0.6 x 2.2: 1 -3.81,-2.6; 2 -2.54,-2.6; 3 -1.27,-2.6; 4 0,-2.6; 5 1.27,-2.6; 6 2.54,-2.6; 7 3.81,-2.6; 8 3.81,2.6; 9 2.54,2.6; 10 1.27,2.6; 11 0,2.6; 12 -1.27,2.6; 13 -2.54,2.6; 14 -3.81,2.6
SO08 = smd 0.6 x 2.2: 1 -1.905,-2.6; 2 -0.635,-2.6; 3 0.635,-2.6; 4 1.905,-2.6; 5 1.905,2.6; 6 0.635,2.6; 7 -0.635,2.6; 8 -1.905,2.6
22-23-2021 = drill 1.067 long: 1 -1.27,0; 2 1.27,0
1210 = smd 1.2 x 2.8: P$1 -1.65,0; P$2 1.65,0
BITECH23B = smd 1.3 x 1.3: 1 1.15,-2.75; 3 -1.15,-2.75 | smd 2 x 1.3: 2 0,2.75
TO-220 = drill 1.067 long: 1 -2.54,0; 2 0,0; 3 2.54,0
HEADER2ROW1POS = drill 0.889 octagon: 1A -1.27,0; 1B 1.27,0
SOT-23 = smd 1 x 1.4: 1 -0.95,-1.1; 2 0.95,-1.1; 3 0,1.1
DIL16 = drill 0.889 long: 1 -8.89,-3.81; 2 -6.35,-3.81; 3 -3.81,-3.81; 4 -1.27,-3.81; 5 1.27,-3.81; 6 3.81,-3.81; 7 6.35,-3.81; 8 8.89,-3.81; 9 8.89,3.81; 10 6.35,3.81; 11 3.81,3.81; 12 1.27,3.81; 13 -1.27,3.81; 14 -3.81,3.81; 15 -6.35,3.81; 16 -8.89,3.81
TESTPT4952 = drill 1.321: P$1 0,0
HEADER2ROW2POS = drill 0.889 octagon: 1A -1.27,1.27; 1B 1.27,1.27; 2A -1.27,-1.27; 2B 1.27,-1.27
HEADER2ROW3POS = drill 0.889 octagon: 1A -1.27,1.27; 1B 1.27,1.27; 2A -1.27,-1.27; 2B 1.27,-1.27; 3A -1.27,-3.81; 3B 1.27,-3.81

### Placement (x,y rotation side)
BIASPOT  35.84,27.58 180 bottom
C1  30.12,6.93 90 top
C2  45.95,7.95 180 top
C3  35.92,7.11 90 top
C4  4.45,17.78 90 bottom
C5  11.2,17.6 270 bottom
C6  14.58,10.85 0 top
C7  14.58,18.49 180 top
C8  17.25,53.34 0 top
C9  6.76,63.47 270 top
C10  22.94,64.54 180 top
C11  12.45,56.72 90 top
C12  14.58,51.38 0 bottom
C13  105.26,3.2 0 top
C14  46.76,54.76 270 top
C15  41.43,42.14 270 top
C16  101.35,20.45 90 top
C17  106.68,5.33 0 top
C18  11.02,12.45 90 top
C19  8.71,17.42 90 top
C20  121.21,47.88 0 top
C21  106.68,31.29 180 bottom
C22  74.93,23.85 90 top
C23  61.62,10.31 270 top
C25  71.12,40.89 90 top
C27  78.77,48.9 0 top
C28  91.21,56.72 0 top
C29  75.21,61.52 270 top
C30  79.48,40.54 90 top
C31  68.81,43.56 270 top
C32  34.49,49.25 0 top
C33  31.83,36.09 90 top
C34  112.01,53.34 180 top
C35  119.13,33.43 270 top
C36  66.14,39.47 90 top
C37  78.59,52.81 0 top
C38  47.29,12.98 90 top
C40  57.25,20.45 90 top
C41  73.08,17.78 90 top
C44  49.25,57.61 90 top
C45  49.61,42.49 90 top
C46  24.18,46.05 270 top
C47  27.74,56.36 270 top
C48  88.9,62.23 270 top
C49  114.15,31.47 0 bottom
C50  33.43,6.76 270 top
C51  30.23,18.85 180 top
C52  40.54,17.78 180 top
CURFEEDBACK  59.03,73.43 0 bottom
CURRENT_FEEDFORWARD  42.49,73.43 0 bottom
D1  18.67,18.31 90 top
D2  18.85,10.85 90 top
D3  13.51,73.08 90 top
D4  15.82,73.08 270 top
D5  109.17,60.81 270 top
D6  112.37,58.85 180 top
D7  13.51,68.63 90 top
D8  15.82,68.63 270 top
ERROFFSETPOT  27.05,27.53 180 bottom
ERRORIN  75.56,73.43 0 bottom
FASTERRORIN  25.96,73.43 0 bottom
FASTOUT  9.42,73.43 0 bottom
IC1  103.12,10.85 0 top
IC2  119.66,61.52 180 top
INTONLED  125.17,33.96 90 bottom
INTRESETBNC  108.28,22.58 0 bottom
INTRESETSWITCH  116.1,22.58 0 bottom
L1  14.58,13.51 180 top
L2  14.58,16.36 180 top
LOCKLED  125.17,25.43 90 bottom
POWIN  5.69,10.67 180 bottom
PZT_OUT1  92.1,73.43 0 bottom
PZTFEEDFORWARD  125.17,73.43 0 bottom
R1  40.54,21.69 0 top
R2  40.54,19.56 0 top
R3  12.98,53.34 180 top
R4  4.98,59.21 90 bottom
R5  19.38,68.81 180 top
R6  25.25,56.36 270 top
R7  9.78,63.47 90 top
R8  76.81,57.96 180 top
R9  81.25,55.47 180 top
R10  109.88,55.47 180 top
R11  127.13,19.74 270 bottom
R12  109.52,27.03 90 top
R13  111.48,27.03 90 top
R14  113.26,40.89 90 top
R15  107.39,27.03 90 top
R16  127.84,41.43 270 top
R17  115.39,41.07 90 top
R18  7.11,68.45 0 top
R19  8.18,40.54 90 top
R20  44.63,54.76 90 top
R21  43.38,42.14 270 top
R22  25.25,38.23 180 top
R23  26.31,46.05 270 top
R24  95.15,40.49 90 top
R25  25.25,40.18 180 top
R26  82.14,5.69 270 top
R27  98.68,46.58 180 top
R28  55.3,35.38 0 top
R29  59.56,42.49 270 bottom
R30  85.88,67.74 0 top
R31  121.26,53.16 0 top
R32  121.26,51.21 180 top
R33  111.84,38.05 0 top
R34  112.9,64.9 90 top
R35  118.95,29.87 0 bottom
R36  15.44,44.83 270 bottom
R37  125.7,41.43 90 top
R38  43.92,18.52 270 top
R39  46.23,18.49 270 top
R40  49.43,12.98 270 top
R41  68.43,7.92 90 top
R42  68.28,29.69 90 top
R43  72.54,4.01 0 top
R44  74.68,50.5 0 top
R45  46.76,42.49 90 top
R46  75.29,17.83 90 top
R47  110.77,5.33 0 top
R48  105.97,16.54 0 top
R49  36.98,31.11 0 top
R50  71.83,67.56 0 top
R51  96.37,8.53 0 top
R52  96.19,62.94 180 top
R53  121.97,70.41 180 top
R54  64.19,26.31 180 top
R55  59.74,20.45 90 top
R56  86.59,62.23 270 top
R57  73.07,16.36 270 bottom
R58  115.93,59.92 90 top
R59  48.18,25.78 180 bottom
R60  18.67,27.56 270 bottom
R63  83.74,73.25 180 top
R64  55.3,69.7 180 top
R65  86.23,71.3 0 top
R66  20.8,57.07 180 top
R67  14.94,56.36 90 top
R69  100.28,36.09 270 bottom
R70  96.9,15.82 180 top
R71  60.81,69.7 0 top
R72  93.7,14.94 90 top
R73  96.01,20.8 0 bottom
R74  109.7,70.23 180 top
R75  97.43,30.76 270 bottom
R76  19.77,48.54 270 bottom
RAMPIN  108.64,73.43 0 bottom
RESETSWITCH  122.33,41.61 90 bottom
U1  40.36,13.51 270 top
U3  17.07,60.99 270 top
U4  65.79,19.2 270 top
U5  108.25,47.5 90 top
U6  75.56,43.56 180 top
U8  81.97,61.16 180 top
U10  35.38,43 270 top
U11  110.41,34.85 180 bottom
U12  32.18,13.16 0 top
U$1  65.61,12.09 90 bottom
U$2  86.23,39.12 90 top
U$3  86.23,46.76 90 top
U$4  52.27,21.69 90 bottom
U$5  20.27,43.56 0 bottom
U$6  122.5,19.2 180 bottom
U$7  119.3,34.14 270 bottom
U$8  58.85,56.72 270 bottom
X1  59.21,15.82 0 bottom
X2  13.87,4.45 180 bottom
X3  50.85,33.43 180 bottom
X4  94.95,67.03 180 bottom
X5  5.87,44.81 180 bottom
X6  11.2,48.36 0 bottom
X7  5.16,52.1 0 bottom
X8  15.29,35.03 180 bottom
X9  27.2,35.38 0 bottom
X10  40.89,48.72 0 bottom
X11  96.37,37.16 0 bottom
X12  40.18,36.98 0 bottom
X13  20.24,32.84 0 bottom
X14  59.74,28.09 0 bottom
X15  24.54,16.36 0 bottom
X16  24,10.67 0 bottom
X17  78.38,4.99 90 bottom
X18  55.47,40.36 0 bottom
X19  23.47,21.87 0 bottom
X20  11.76,41.96 0 bottom
X21  80.19,11.2 270 bottom
X22  5.51,26.31 0 bottom
X23  37.41,63.58 0 bottom
X24  6.05,35.74 270 bottom
X25  80.72,17.07 180 bottom
X26  35.92,57.07 180 bottom
X27  28.09,61.52 0 bottom
X34  51.79,8.46 0 bottom
X35  60.81,38.23 0 bottom
X36  66.5,52.27 0 bottom
X38  71.12,53.16 0 bottom
X42  71.42,10.9 270 bottom
X43  69.55,25.12 0 bottom
X44  5.51,30.94 0 bottom
X47  102.41,66.67 0 bottom
X48  100.99,59.74 0 bottom
X50  87.12,50.67 0 bottom

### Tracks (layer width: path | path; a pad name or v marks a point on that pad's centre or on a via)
+5V  (via drill 0.51)
  Top 0.178: R33.2 112.95,38.05 U11.3 112.95,31.83 105.79,31.83 105.79,35.74 102.23,35.74 102.23,32.54 v90.68,32.54 | 83.74,48.67 U$3.5 85.34,48.67 85.34,40.89 83.63,40.89 U$2.5 82.5,41.02 v82.5,41.96 | R16.2 127.84,29.34 120.19,29.34 v120.19,27.2 | 122.33,53.16 R31.2 v124.64,53.16
  Bottom 0.178: C49.2 112.95,31.47 | 118.64,27.2 v120.19,27.2 | v82.5,41.96 90.68,41.96 v90.68,32.54 | v124.64,53.16 116.1,53.16 116.1,34.85 U11.3
  Bottom 0.406: 117.35,27.74 118.64,27.74 118.64,27.2 INTRESETSWITCH.1 118.77,22.58 118.77,18.14 122.5,18.14 U$6.3 | 117.35,27.74 113.26,27.74 113.26,31.47 C49.2 113.05,34.85 U11.3 | R35.P$2 117.35,29.87 117.35,27.74
+15V  (via drill 0.51, 0.51 pad 0.51, 0.71 pad 0.51)
  Top 0.178: 40.36,7.64 44.85,7.64 | 40.36,7.64 40.36,15.42 42.85,15.42 | 42.85,15.42 U1.8 | v80.72,27.56 80.72,27.57 83.92,27.57 83.92,33.78 86.94,33.78 86.94,40.89 91.21,40.89 | U6.8 77.34,40.96 v77.34,38.58 79.48,38.58 C30.1 | 91.21,40.89 91.21,48.67 U$3.4 90.14,48.67 v90.14,50.67 | 91.21,40.89 88.83,40.89 U$2.4 | 83.87,58.5 v90.14,58.5 90.14,56.72 C28.1 | 20.27,64.54 C10.2 | 30.12,8 C1.2 | 30.12,8 31.47,8 | 31.47,8 31.47,10.56 U12.2 | 42.85,15.42 42.85,15.65 | IC2.7 120.19,58.92 120.19,56.01 127.48,56.01 127.48,46.23 | R24.1 100.28,39.39 v100.28,38.94 | U10.8 37.98,47.3 35.92,47.3 | C32.2 35.59,47.3 35.92,47.3 | v30.4,47.3 35.92,47.3 | 1.6,39.65 v4.45,39.65 | 30.12,8 24,8 X16.P$1 | 31.47,8 31.47,4.09 40.36,4.09 40.36,7.64 | C22.1 75.03,22.75 75.03,21.11 | 103.12,1.07 103.12,3.02 | 103.12,3.02 IC1.4 | C13.1 103.12,3.2 103.12,3.02
  Top 0.406: 21.34,12.8 21.34,7.82 | 21.34,7.82 21.34,1.07 84.45,1.07 | 84.45,1.07 91.75,1.07 | 91.75,1.07 103.12,1.07 129.62,1.07 129.62,46.23 127.48,46.23 119.84,46.23 | C2.2 44.85,7.64 43.56,7.64 | X16.P$1 24,12.8 21.34,12.8 | 21.34,12.8 21.34,12.85 D2.1 18.85,13.51 L1.1 C6.2 15.68,8.89 v14.76,8.89 14.76,7.47 11.2,7.47 11.2,4.45 X2.1 | 91.75,1.07 91.57,1.07 | 119.84,46.23 U5.3 108.99,46.23 108.99,38.94 107.87,38.94 | C20.1 119.84,47.88 119.84,46.23 | 107.87,38.94 v100.28,38.94 | 21.34,7.82 21.34,1.42 | U3.8 20.27,62.89 20.27,64.54 v20.27,65.61 | v1.6,22.58 1.6,39.65 1.6,65.61 v2.49,65.61 | 83.87,58.5 U8.8 | 107.87,38.94 U11.1 | 72.36,21.11 75.03,21.11 84.45,21.11 84.45,1.07 | 72.36,21.11 U4.8 | 72.36,21.11 v72.36,23.29
  Bottom 0.178: v80.72,27.56 80.72,25.43 72.36,25.43 72.36,38.58 v77.34,38.58 | v90.14,50.67 v90.14,58.5 | 107.87,31.29 C21.2 107.78,34.85 U11.1 | v100.28,38.94 R69.1 | v30.4,47.3 30.4,39.65 v4.45,39.65
  Bottom 0.406: v1.6,22.58 14.76,22.58 v14.76,8.89 | v2.49,65.61 v20.27,65.61 | v72.36,23.29 72.36,25.43
-15V  (via drill 0.51, 0.51 pad 0.51)
  Top 0.178: 37.76,8.21 U1.4 | 37.76,8.21 C3.2 37.87,8.21 v37.87,7.11 | 37.76,8.21 37.76,8.18 37.87,8.18 | 61.55,12.45 C23.1 | 68.81,46.16 63.48,46.16 63.48,32.77 | 68.81,46.16 U6.4 73.61,46.16 v73.61,48.54 | U$3.7 83.63,46.05 v81.25,46.05 | v81.25,38.58 83.63,38.58 U$2.7 | 68.81,46.16 C31.1 | 75.39,63.76 69.52,63.76 v69.52,48.72 | 75.39,63.76 U8.4 | C29.1 75.39,62.62 75.39,63.76 | 12.45,59.08 C11.2 | IC2.4 117.88,64.12 v117.88,66.67 | U10.4 32.78,38.76 v31.83,38.76 C33.2 | 61.55,12.45 56.19,12.45 56.19,12.38 | U4.4 63.19,12.45 61.55,12.45 | IC1.11 102.95,13.45 102.95,17.78 101.35,17.78 | 101.35,17.78 85.52,17.78 v85.52,16.36 | 101.35,17.78 C16.1
  Top 0.406: C7.1 L2.1 18.67,16.36 D1.2 21.34,16.31 v21.34,16.36 21.34,21.87 X19.P$1 | 63.48,32.77 56.19,32.77 v56.19,31.83 | U3.4 12.45,59.08 10.31,59.08 v10.31,59.03 | 56.19,12.62 56.19,12.45 | 56.19,12.62 v56.19,13.34 | 56.19,12.62 v56.19,2.13 56.19,1.96
  Bottom 0.178: v81.25,38.58 v81.25,46.05 81.25,50.14 73.61,50.14 v73.61,48.54 73.61,48.72 v69.52,48.72 | 2.49,32.89 2.49,32.72 | 2.49,24.89 2.49,25.07 | v117.88,66.67 129.79,66.67 129.79,41.78 129.69,41.78 | 2.49,38.76 v31.83,38.76 | v37.87,7.11 | 37.87,1.99 v37.87,7.11 | 85.52,1.96 v85.52,16.36
  Bottom 0.406: 21.34,2.01 37.87,1.99 55.83,1.96 | 55.83,1.96 57.78,1.96 85.52,1.96 129.69,1.96 129.69,41.78 | 21.34,2.01 v21.34,16.36 | 55.83,1.96 v56.19,2.13 | X19.P$1 23.47,23.29 2.49,23.29 2.49,24.89 2.49,32.89 2.49,38.76 2.49,59.03 v10.31,59.03 | v56.19,13.34 v56.19,31.83 | v56.19,2.13 | X2.3 18.67,4.45 18.67,1.96 21.34,1.96 21.34,2.01
CURRERRSIG
  Top 0.178: C44.P$1 49.25,53.66 C14.2
  Bottom 0.178: C44.P$1 50.85,53.8 50.85,54.76 52.63,54.76 52.63,57.96 55.04,57.96 U$8.13 U$8.14
ERR_OFFSET  (via drill 0.51)
  Top 0.178: 43.74,19.62 R38.1 v43.92,21.51 | v32.18,31.29 22.58,31.29 22.58,30.23 10.31,30.23 10.31,30.94 9.86,30.94 | 9.86,30.94 X44.P$1 | X24.1B X24.2B X24.3B 9.86,30.94
  Bottom 0.178: v43.92,21.51 43.92,31.29 v32.18,31.29
ERRORSIG  (via drill 0.51)
  Top 0.178: v71.83,59.21 71.83,58.14 75.71,58.14 R8.2
  Bottom 0.178: v71.83,59.21 65.96,59.21 65.96,60.45 62.66,60.45 U$8.3 64.72,60.53 64.72,65.61 | 64.72,65.61 U$8.1 | ERRORIN.INCOND 73.61,73.43 73.61,71.48 64.72,71.48 64.72,65.61
FASTERROR-  (via drill 0.51 pad 0.51)
  Top 0.178: v20.09,53.34 C8.2 18.35,51.38 C12.P$1
  Bottom 0.178: v20.09,53.34 24,53.34 24,59.92 26.82,59.92 X27.2B X27.1B
FASTERROROUT
  Top 0.178: FASTOUT.INCOND 8.71,73.43 | R18.P$2 11.38,68.45 11.38,70.23 13.51,70.23 D7.2 D3.1
  Top 0.406: FASTOUT.INCOND 8.76,73.43 R18.P$2
GND  (via drill 0.51, 0.51 pad 0.51)
  Top 0.178: 22.29,16.36 24.29,16.36 | 24.29,16.36 X15.P$1 | 24.64,13.79 24.64,18.74 | 24.29,16.36 26.54,16.36
  Top 0.406: 14.76,11.84 14.76,11.73
  other vias: 111.84,18.14 77.52,43.03 73.43,37.34 66.67,40.36 86.94,56.72 88.01,53.87 72.54,61.16 11.91,8.71 22.4,59.21 10.31,56.36 114.86,52.1 103.12,50.67 102.77,46.05 102.77,42.67 29.34,49.61 16.18,64.36 8.89,26.67 12.8,21.34 27.74,13.34 35.2,13.16 42.14,9.78 39.12,9.42 35.74,22.94 37.16,39.12 34.14,39.29 28.8,41.78 78.77,61.16 85.17,59.56 86.59,46.76 85.7,38.05 82.14,32.36 70.59,32.36 124.82,49.78 123.57,61.34 114.68,62.59 43.92,65.43 39.83,59.03 18.67,64.36 21.51,54.41 16.54,56.36 14.05,49.78 20.8,36.45 50.32,49.43 46.94,34.67 43.74,37.87 45.16,25.6 41.78,25.6 54.76,4.62 19.74,5.16 22.94,3.56 5.69,40.72 7.82,49.61 30.76,55.12 30.05,66.32 32.72,66.32 90.5,25.25 93.7,25.25 86.59,4.27 95.12,54.41 95.12,47.65 94.41,58.85 90.68,60.27 7.29,57.25 64.01,8.36 58.14,4.45 70.59,36.8 72.54,40.89 68.99,13.87 65.79,17.42 40.01,54.76 43.56,45.69 8.53,29.87 15.65,31.83 11.91,37.34
  pour Top: 0,82.37 0,0 132.11,0 132.11,82.37
  pour Bottom: -0.36,82.37 0,0 132.11,0 131.75,82.37
INT2A  (via drill 0.51 pad 0.51)
  Top 0.178: v83.39,43.2 76.1,44.45 76.1,46.16 U6.2 76.2,48.9 C27.1 77.52,48.9 77.52,50.49 R44.2 75.92,50.49 75.92,52.81 C37.P$1 | v88.9,43.2 88.83,43.2 U$3.1
  Bottom 0.178: v83.39,43.2 v88.9,43.2 | C37.P$1 71.12,52.81 X38.P$1
INT2B  (via drill 0.51)
  Top 0.178: 79.83,46.16 U6.1 | 79.83,46.16 80.01,46.16 80.01,44.81 83.63,44.81 U$3.8 | 79.83,46.16 79.83,48.9 C27.2 81.25,48.9 81.25,52.81 | 81.25,52.81 C37.P$2 | v73.61,56.54 73.79,56.54 73.79,54.59 78.23,54.59 78.23,52.81 81.25,52.81 | v67.21,57.61 65.96,57.61 65.96,56.72 60.45,56.72 60.45,47.83 U$8.8
  Bottom 0.178: 82.4,51.03 82.4,50.85 | C37.P$2 82.4,51.03 | X50.P$1 82.4,50.67 82.4,51.03 | v73.61,56.54 67.21,56.54 v67.21,57.61
INTA  (via drill 0.51 pad 0.51)
  Top 0.178: U$2.1 89.08,37.21 v89.08,34.85 | v82.14,34.85 82.14,36.27 75.03,36.27 75.03,38.41 | 68.45,35.66 C36.P$1 | 68.45,35.66 68.63,35.66 68.63,39.83 71.12,39.83 C25.1 | C25.1 70.41,39.83 | R42.2 68.45,30.79 68.45,35.66 | U6.6 75.03,40.96 75.03,38.41 | C25.1 70.94,39.79 70.94,38.41 75.03,38.41
  Bottom 0.178: v82.14,34.85 v89.08,34.85 | C36.P$1 66.14,38.23 X35.P$1
INTB  (via drill 0.51 pad 0.51)
  Top 0.178: U$2.8 83.63,37.16 76.1,37.16 76.1,40.96 U6.7 76.2,42.85 72.36,42.85 | v72.19,44.81 72.36,44.81 72.36,42.85 | 72.36,42.85 71.12,42.85 C25.2 | U$8.5 U$8.6 66.5,52.91 X36.P$1
  Bottom 0.178: 67.39,44.81 67.03,44.81 C36.P$2 66.14,43.2 | 67.39,44.81 v72.19,44.81 | 67.39,44.81 67.39,48.9 | 67.39,48.9 67.39,49.05 | X36.P$1 66.5,49.07 67.39,49.07 67.39,48.9
INTOUT  (via drill 0.51)
  Top 0.178: 70.73,65.25 R50.1 | 70.73,65.25 77.17,65.25 v77.17,67.03 | U$8.9 55.04,50.32 | 70.73,65.25 65.96,65.25 65.96,64.36 59.38,64.36 59.38,50.32 55.04,50.32 | 55.04,50.32 U$8.10 | D5.1 109.17,63.8 108.81,63.8 v108.81,65.96 112.9,65.96 R34.2
  Bottom 0.178: v77.17,67.03 77.17,71.12 79.3,71.12 79.3,72.54 83.03,72.54 83.03,69.88 108.81,69.88 v108.81,65.96 | U$8.9 55.12,47.83 55.12,44.27 59.56,44.27 R29.1
LIMIT_TTL  (via drill 0.51)
  Top 0.178: R14.2 113.26,43.74 110.86,43.74 U5.1 110.86,38.05 R33.1 109.17,38.05 v109.17,37.34 | v103.66,34.67 103.66,25.96 103.83,25.96 | 103.83,25.96 107.39,25.96 R15.1 | v121.61,22.05 121.61,19.38 103.83,19.38 103.83,25.96
  Bottom 0.178: v109.17,37.34 103.66,37.34 v103.66,34.67 | U$6.1 121.61,20.3 v121.61,22.05
N$1
  Top 0.178: 9.96,61.7 9.96,62.38 R7.1 C9.2 | 9.96,61.7 14.47,61.7 U3.2 | 9.96,61.7 9.07,61.7 9.07,55.65 | 9.07,53.34 9.07,55.65 | 9.07,53.34 R3.2 | 9.07,48.36 9.07,53.34 | 9.07,48.36 X6.P$1 | R4.P$1 9.07,55.4 9.07,55.65 | X5.2 9.07,44.81 9.07,48.36
N$2
  Top 0.178: U1.2 39.47,14.15 39.47,16.54 41.64,16.54 C52.1 R2.2 R1.2
N$3
  Top 0.178: C8.1 R3.1 14.08,51.38 C12.P$2
N$4
  Top 0.178: R22.1 R25.1 26.35,43.56 | R22.1 26.35,38.12 | 26.35,43.64 U10.2 | 26.35,43.56 26.35,43.64 | 22.94,43.56 U$5.1A 21.54,40.89 18.31,40.89 18.31,35.03 X8.2 | 22.94,43.56 26.35,43.56 | 26.35,43.64 26.35,44.95 R23.2 C46.2 | X9.P$1 26.35,35.38 R22.1 | 22.94,43.56 22.94,53.7 34.65,53.7 X26.1A
N$5
  Bottom 0.178: R69.2 100.18,34.99 R75.3
N$6
  Top 0.178: C9.1 6.76,64.72 | 4.98,64.58 3.2,64.58 3.2,52.09 X7.P$1 5.16,44.81 X5.1 | 4.98,64.58 5.33,64.58 | 4.98,64.58 R4.P$2
  Top 0.406: R18.P$1 5.33,68.45 5.33,64.58 C9.1 R7.2 9.78,64.54 14.4,64.54 14.4,62.89 U3.1
N$7
  Top 0.178: R5.2 17.42,68.81 17.42,60.27 17.6,60.27 | 17.6,60.27 19.67,60.27 U3.6 | 17.6,60.27 17.6,55.26 R6.2 C47.2
N$8
  Top 0.178: FASTERRORIN.INCOND 24.71,73.43 24.71,68.81 R5.1
  Bottom 0.178: FASTERRORIN.INCOND 24.82,68.81 31.47,68.81 31.47,60.25 X27.2A
N$9  (via drill 0.51 pad 0.51)
  Top 0.178: U3.7 22.4,61.62 22.4,61.7 v23.11,61.7 24.71,61.7 24.71,61.52 | C47.1 R6.1 24.71,57.46 24.71,61.52 | X27.1A 29.34,62.79 29.34,61.52 24.71,61.52
N$10
  Top 0.178: INTRESETBNC.1 109.53,22.58 R12.1
N$11
  Bottom 0.406: INTONLED.2 122.33,35.23 122.33,33.07 120.4,33.07 U$7.2
N$12
  Top 0.178: 111.48,25.6 116.1,25.6 INTRESETSWITCH.2
  Top 0.406: R13.1 111.48,25.6
N$13  (via drill 0.51)
  Top 0.178: v120.37,36.45 120.37,37.69 125.7,37.69 R37.1
  Bottom 0.178: U$7.1 120.37,35.09 v120.37,36.45
N$14
  Top 0.178: C50.1 33.43,8 32.72,8 32.72,10.56 U12.3
N$15
  Top 0.178: U8.6 81.25,58.56 81.25,56.72 80.16,56.72 R9.2 80.16,56.01 78.23,56.01 78.23,57.96 R8.1
N$16  (via drill 0.51)
  Top 0.178: 108.28,53.34 C34.2 110.91,51.31 U5.7 | v106.15,40.54 108.28,40.54 108.28,53.34 | 108.28,53.34 108.78,53.34 R10.2 | v111.66,39.83 111.66,39.79 R14.1 113.26,39.97 R17.1
  Bottom 0.178: v111.66,39.83 106.15,39.83 v106.15,40.54
N$17  (via drill 0.51)
  Top 0.178: R13.2 117.88,28.13 117.88,34.67 | 117.88,34.67 v117.88,38.94 | C35.1 117.88,34.53 117.88,34.67 | U5.5 117.88,48.77 v117.88,47.65
  Top 0.406: R13.2 R12.2 R15.2
  Bottom 0.178: v117.88,38.94 v117.88,47.65
N$18
  Top 0.178: R17.2 116.64,42.88 RESETSWITCH.2
N$19
  Top 0.178: R45.P$2 46.76,43.2 46.41,43.2 46.41,43.24 R21.1 C15.1 41.25,43.24 41.25,43.92 37.98,43.92 U10.7 35.74,43.64 35.74,32.72 24.15,32.72 | 24.15,32.72 R22.2 | 24.15,32.72 20.24,32.72 X13.P$1
  Bottom 0.178: R45.P$2 C45.P$2
N$20  (via drill 0.51)
  Top 0.178: 26.31,47.3 v26.31,51.38 41.07,51.38 | 26.31,47.3 28.27,47.3 28.27,44.91 | 28.27,44.91 28.27,44.81 | 28.27,44.91 U10.1 | 26.31,47.3 R23.1 C46.1 | R64.2 42.67,69.7 42.67,51.38 41.07,51.38 | X10.P$1 41.07,48.72 41.07,51.38 | v16.89,41.43 16.89,37.87 14.02,37.87 X8.1
  Bottom 0.178: v26.31,51.38 20.09,51.38 20.09,49.25 16.27,49.25 R76.2 16.27,47.47 15.44,47.47 | R36.1 15.65,45.93 | R36.1 15.44,45.52 | v16.89,41.43 16.89,45.87 15.44,45.87 R36.1 | 15.44,47.47 v13.87,47.47 | R36.1 15.44,47.47 | X26.2A 35.92,58.34 35.92,53.34 38.76,53.34 38.76,48.72 X10.P$1
N$21
  Top 0.178: 73.08,18.93 C41.2 | 73.08,18.93 R46.2 79.45,18.93 X25.2A | 73.08,19.84 73.08,18.93 | 73.08,19.84 73.15,19.84 | 73.08,19.84 U4.7 66.32,19.84 66.32,26.31 | 66.32,26.31 R54.1 | 66.32,26.31 68.28,26.31 | 68.28,26.31 R42.1 | X43.P$1 68.28,25.12 68.28,26.31
  Bottom 0.178: R57.3 79.45,17.51 X25.2A
N$22
  Top 0.178: C44.P$2 49.25,61.52 46.76,61.52 C14.1 R20.2
N$23
  Top 0.178: C15.2 41.43,41.1 39.65,42.32 37.98,42.32 U10.6 | C15.2 R21.2 46.23,41.04 | 46.23,41.04 46.58,41.04 46.58,41.07 46.76,41.07 R45.P$1 C45.P$1 | R20.1 44.63,49.96 48.18,49.96 48.18,41.04 46.23,41.04 | X12.P$1 41.43,36.98 C15.2
N$24
  Top 0.178: D3.2 D4.1
N$25
  Top 0.178: D7.1 D8.2
N$26
  Top 0.178: R19.1 10.49,39.44 X20.2
N$27  (via drill 0.51)
  Top 0.178: R25.2 24.18,40.18 v24.18,41.6 | v24.18,50.32 24.18,52.63 41.22,52.63 CURRENT_FEEDFORWARD.INCOND
  Bottom 0.178: v24.18,41.6 v24.18,50.32
N$28
  Top 0.178: 82.14,6.76 R26.1 78.38,6.79 X17.2
N$29
  Bottom 0.178: X18.1 59.56,40.36 R29.2
N$30
  Top 0.178: X25.1B 83,15.8 83,10 80.19,10 X21.2
N$31
  Bottom 0.178: R76.1 19,47.39 U$5.1B
N$32
  Bottom 0.178: 15.44,42.49 R36.2 15.44,41.96 X20.1
N$33
  Top 0.178: IC1.1 99.39,8.25 99.39,6.22 100.58,6.22 IC1.2
N$34
  Top 0.178: IC1.7 107.78,8.25 C17.2 R47.1
N$35
  Top 0.178: 73.64,4.22 R43.2 78.38,4.01 X17.1
N$36
  Top 0.178: X18.2 R28.1
N$37
  Top 0.178: ERROFFSETPOT.2 27.05,24.89 15.11,24.89 15.11,28.63 3.02,28.63 3.02,37.01 X24.1A
N$38
  Bottom 0.178: X21.1 83.5,12.47 83.5,18.5 81.99,18.5 X25.2B
N$39  (via drill 0.51)
  Top 0.178: U8.7 82.36,58.56 R9.1 82.36,55.65 v84.81,55.65
  Bottom 0.178: v84.81,55.65 65.25,55.65 65.25,57.96 62.66,57.96 | U$8.2 60.27,63.07 60.27,57.96 62.66,57.96 | 62.66,57.96 U$8.4
N$40  (via drill 0.51)
  Top 0.178: U5.13 105.66,44.81 99.03,44.81 99.03,43.74 v96.9,43.74 95.12,43.74 95.12,41.59 R24.2 | R10.1 112.72,55.47 v112.72,56.19
  Bottom 0.178: v112.72,56.19 93.7,56.19 93.7,43.74 v96.9,43.74
N$41
  Top 0.178: R31.1 R32.2 117.88,51.21 117.88,50.04 U5.6 109.17,50.04 109.17,47.47 110.86,47.47 U5.4
N$42
  Bottom 0.406: U$6.2 124.99,20.3 124.99,18.14 127.13,18.14 R11.P$2
N$43  (via drill 0.51)
  Top 0.178: X11.P$1 92.63,37.16 92.63,50.16 98.32,50.16 v98.32,48.72 | v102.77,48.72 105.66,48.72 U5.10
  Bottom 0.178: v98.32,48.72 v102.77,48.72 | X11.P$1 94.68,37.16 R75.2
N$44
  Top 0.178: X23.2 36,63.58 36,55.75 37.19,55.75 X26.1B
N$45
  Bottom 0.406: LOCKLED.1 127.13,24.16 R11.P$1
N$46
  Top 0.178: R55.1 C40.1 52.27,19.35 U$4.1A 52.27,20.45 54.05,20.45 54.05,24.89 52.09,24.89 52.09,33.43 X3.2 | R55.1 61.52,19.35 61.52,19.74 63.19,19.74 | R54.2 62.76,26.31 62.76,23.11 64.9,23.11 64.9,19.74 63.19,19.74 | 63.19,19.74 U4.2 | X1.P$1 59.74,15.82 R55.1
N$47
  Top 0.178: R38.2 46.23,17.42 R39.2 51.92,17.39 51.92,11.91 49.43,11.91 R40.2 C38.1 47.3,11.61 46.23,11.61 46.23,12.8 42.96,12.8 U1.6
N$48  (via drill 0.51)
  Top 0.178: U1.7 47.3,14.15 C38.2 R40.1 49.61,14.08 v49.61,16 | v58.5,10.49 58.5,6.83 R41.1 71.44,6.83 R43.1
  Bottom 0.178: 54.23,10.49 53.87,10.49 53.87,16 v49.61,16 | 54.23,10.49 v58.5,10.49 | X34.P$1 54.23,8.46 54.23,10.49
N$49
  Top 0.406: C19.1 8.71,16.33 C5.MINUS 13.48,16.33 L2.2
  Bottom 0.406: POWIN.3 8.18,10.67 8.18,16.36 11.2,16.36 C5.MINUS
N$50
  Top 0.406: POWIN.1 3.02,10.67 3.02,16.54 4.45,16.54 C4.PLUS 4.62,16.51 4.62,13.51 11.02,13.51 C18.2 13.48,13.55 L1.2
N$51  (via drill 0.51)
  Top 0.178: D6.2 109.17,58.85 D5.2 v109.17,57.78 | v105.61,57.78 105.08,57.78 105.08,54.41 101.17,54.41 101.17,47.65 | 101.17,47.65 101.17,47.47 105.66,47.47 U5.11 | R27.1 101.17,46.58 101.17,47.65
  Bottom 0.178: v105.61,57.78 v109.17,57.78
N$52
  Bottom 0.178: X23.1 38.75,63.58 38.75,58.25 37.19,58.25 X26.2B
N$53
  Bottom 0.178: U$8.12 59.21,55.45 59.21,50.49 62.66,50.49 U$8.7
N$54
  Bottom 0.178: X24.2A 7.32,35.74 11.73,35.74 11.73,32.18 13.69,32.18 13.69,27.56 R60.2
N$55  (via drill 0.51)
  Top 0.178: R44.1 72.01,50.49 72.01,47.3 65.25,47.3 v65.25,48.54 | U$8.11 55.04,52.98 57.61,52.98 v57.61,52.45
  Bottom 0.178: v57.61,52.45 57.61,49.07 65.25,49.07 v65.25,48.54
N$56
  Bottom 0.178: X47.2 99.75,62.05 98.45,62.05 X48.3
N$59
  Top 0.178: U$1.1A 65.61,10.9 68.45,10.9 | 68.45,10.9 X42.P$1 71.42,17.07 71.48,17.07 | 71.48,17.07 73.08,17.07 C41.1 73.08,16.73 R46.1 75.29,15.8 X25.1A | R41.2 68.45,9.03 68.45,10.9 | 71.48,17.07 71.48,18.49 68.39,18.49 U4.6
N$60
  Bottom 0.178: R57.2 65.61,16.36 U$1.1B
N$62
  Top 0.178: IC1.9 105.66,16.54 R48.1 104.87,18.14 109.17,18.14 109.17,13.16 111.66,13.16 111.66,5.33 R47.2
N$63  (via drill 0.51)
  Top 0.178: R48.2 106.93,16.54 IC1.8 107.04,13.45 107.04,11.91 100.58,11.91 IC1.13 100.64,13.45 v100.64,16
  Bottom 0.178: v100.64,16 99.03,16 99.03,20.8 R73.1
N$64
  Top 0.178: C17.1 105.58,8.25 IC1.6 105.66,10.49 97.61,10.49 97.61,8.53 R51.2
N$65
  Top 0.178: X4.2B X4.1B 97.97,65.76 97.97,68.99 104.95,68.99 X47.1
N$66
  Bottom 0.178: R59.2 52.27,23.03 U$4.1B
N$67
  Top 0.178: PZTFEEDFORWARD.INCOND 123.07,73.43 R53.1
N$68
  Top 0.178: R53.2 112.72,70.41 112.72,75.56 69.34,75.56 69.34,68.81 | 69.34,68.81 73.61,68.81 | 73.61,68.81 82.6,68.81 82.6,67.56 | 82.6,67.56 82.6,65.96 | 82.6,65.96 U8.2 82.6,61.13 R56.2 C48.2 | R50.2 73.61,67.56 73.61,68.81 | R52.2 86.77,66.14 82.6,66.14 82.6,65.96 | R30.1 82.6,67.74 82.6,67.56 | R49.2 42.32,31.11 42.32,34.14 44.27,34.14 44.27,36.63 51.92,36.63 51.92,67.03 69.34,67.03 69.34,68.81
N$69
  Top 0.178: X48.2 100.81,59.74 100.81,62.94 R52.1
N$70
  Bottom 0.406: R35.P$1 125.17,29.87 INTONLED.1
N$72  (via drill 0.51 pad 0.51)
  Top 0.178: v80.54,70.94 80.54,73.25 R63.2 | 85.52,63.86 86.59,63.86 R56.1 C48.1 | v85.52,65.08 85.52,63.86 | 85.52,63.86 83.87,63.86 U8.1
  Bottom 0.178: v80.54,70.94 80.54,65.61 85.52,65.61 v85.52,65.08
N$73
  Top 0.178: 85.17,73.25 R63.1 | 85.17,73.25 85.17,74.5 90.83,74.5 PZT_OUT1.INCOND | 85.17,73.25 85.13,73.25 R65.1
N$74
  Top 0.178: CURFEEDBACK.INCOND 58.14,73.43 58.14,69.7 | R64.1 58.14,69.7 | 58.14,69.7 R71.1
N$75
  Top 0.178: 95.8,13.45 IC1.14 | 95.8,13.45 R70.2 | R51.1 95.8,8.53 95.8,13.45
N$76
  Top 0.178: U3.5 19.7,59.08 R66.2
N$77
  Top 0.178: U3.3 16.36,60.35 16.36,57.43 14.94,57.43 R67.2
N$78
  Top 0.178: 101.73,13.45 IC1.12 101.88,13.45 101.88,17.25 98,17.25 98,17.07 | R72.2 93.7,17.07 98,17.07 | 98,17.07 R70.1
N$80
  Top 0.178: R34.1 116.81,63.8 116.81,62.23 | 116.81,62.23 120.29,62.23 IC2.2 | R58.2 116.81,61.02 116.81,62.23
N$81
  Top 0.178: D6.1 115.93,58.85 R58.1 116.1,58.82 116.1,56.72 119.02,56.72 IC2.6
N$82
  Top 0.178: X4.2A 93.67,71.12 105.94,71.12 RAMPIN.INCOND
N$83
  Bottom 0.178: X4.1A 92.63,65.76 92.63,20.8 R73.2
N$84
  Top 0.178: RAMPIN.OUTCOND 109.85,73.25 R74.2
PROPOUT  (via drill 0.51, 0.51 pad 0.51)
  Top 0.178: R30.2 90.32,67.74 v90.32,65.96 | R55.2 C40.2 57.25,27.03 | R55.2 63.19,21.55 U4.1 | v54.05,27.03 57.25,27.03 | v60.98,23.82 59.74,23.82 R55.2 | X14.P$1 59.74,27.03 57.25,27.03
  Bottom 0.178: v90.32,65.96 91.92,65.96 91.92,22.23 60.98,22.23 v60.98,23.82 | X3.1 49.33,33.43 R59.1 54.05,28.53 v54.05,27.03
PZT_BIAS
  Top 0.178: BIASPOT.2 35.88,27.58 R49.1
PZTERRSIG
  Top 0.178: R39.1 46.41,19.59 46.41,23.29 43.03,23.29 43.03,33.43 44.98,33.43 44.98,35.92 52.63,35.92 52.63,63.07 U$8.15
  Bottom 0.178: U$8.15 U$8.16
TTL_RESET  (via drill 0.51 pad 0.51)
  Top 0.178: U$2.6 83.63,39.83 85.7,39.83 85.7,49.61 | 85.7,49.61 85.7,52.63 v95.12,52.63 | v102.41,52.63 107.21,52.63 107.21,68.28 128.55,68.28 v128.55,48.18 | U5.2 127.66,44.96 127.66,44.45 | v128.55,44.45 127.66,44.45 | U$3.6 81.97,47.4 81.97,49.61 85.7,49.61 | R37.2 R16.1 127.84,44.45 127.66,44.45
  Bottom 0.178: v95.12,52.63 v102.41,52.63 | v128.55,48.18 v128.55,44.45
V+
  Top 0.178: 33.07,15.76 U12.6 32.82,18.85 32.54,18.85 | 32.54,18.85 C51.1 | BIASPOT.3 39.44,27.58 R1.1 32.54,21.69 | 32.54,21.69 32.54,18.85 | ERROFFSETPOT.3 29.69,27.53 29.69,21.69 32.54,21.69
  Bottom 0.178: 18.59,24.71 29.59,24.71 ERROFFSETPOT.3 | 18.59,24.71 18.59,28.89 21.42,28.89 R60.3 | 18.59,24.71 5.51,24.71 X22.P$1
V-  (via drill 0.51)
  Top 0.178: v34.31,19.56 R2.1 C52.2 37.76,17.78 U1.1 | BIASPOT.1 31.47,27.58 31.47,30.23 24.51,30.23 ERROFFSETPOT.1
  Bottom 0.178: BIASPOT.1 33.43,27.58 33.43,22.58 34.31,22.58 v34.31,19.56 | ERROFFSETPOT.1 24.54,27.53 24.54,26.49 21.95,26.49 21.95,26.41 R60.1

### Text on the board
Bottom: DCM 2011 | LASER LOCK | REV 1.1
